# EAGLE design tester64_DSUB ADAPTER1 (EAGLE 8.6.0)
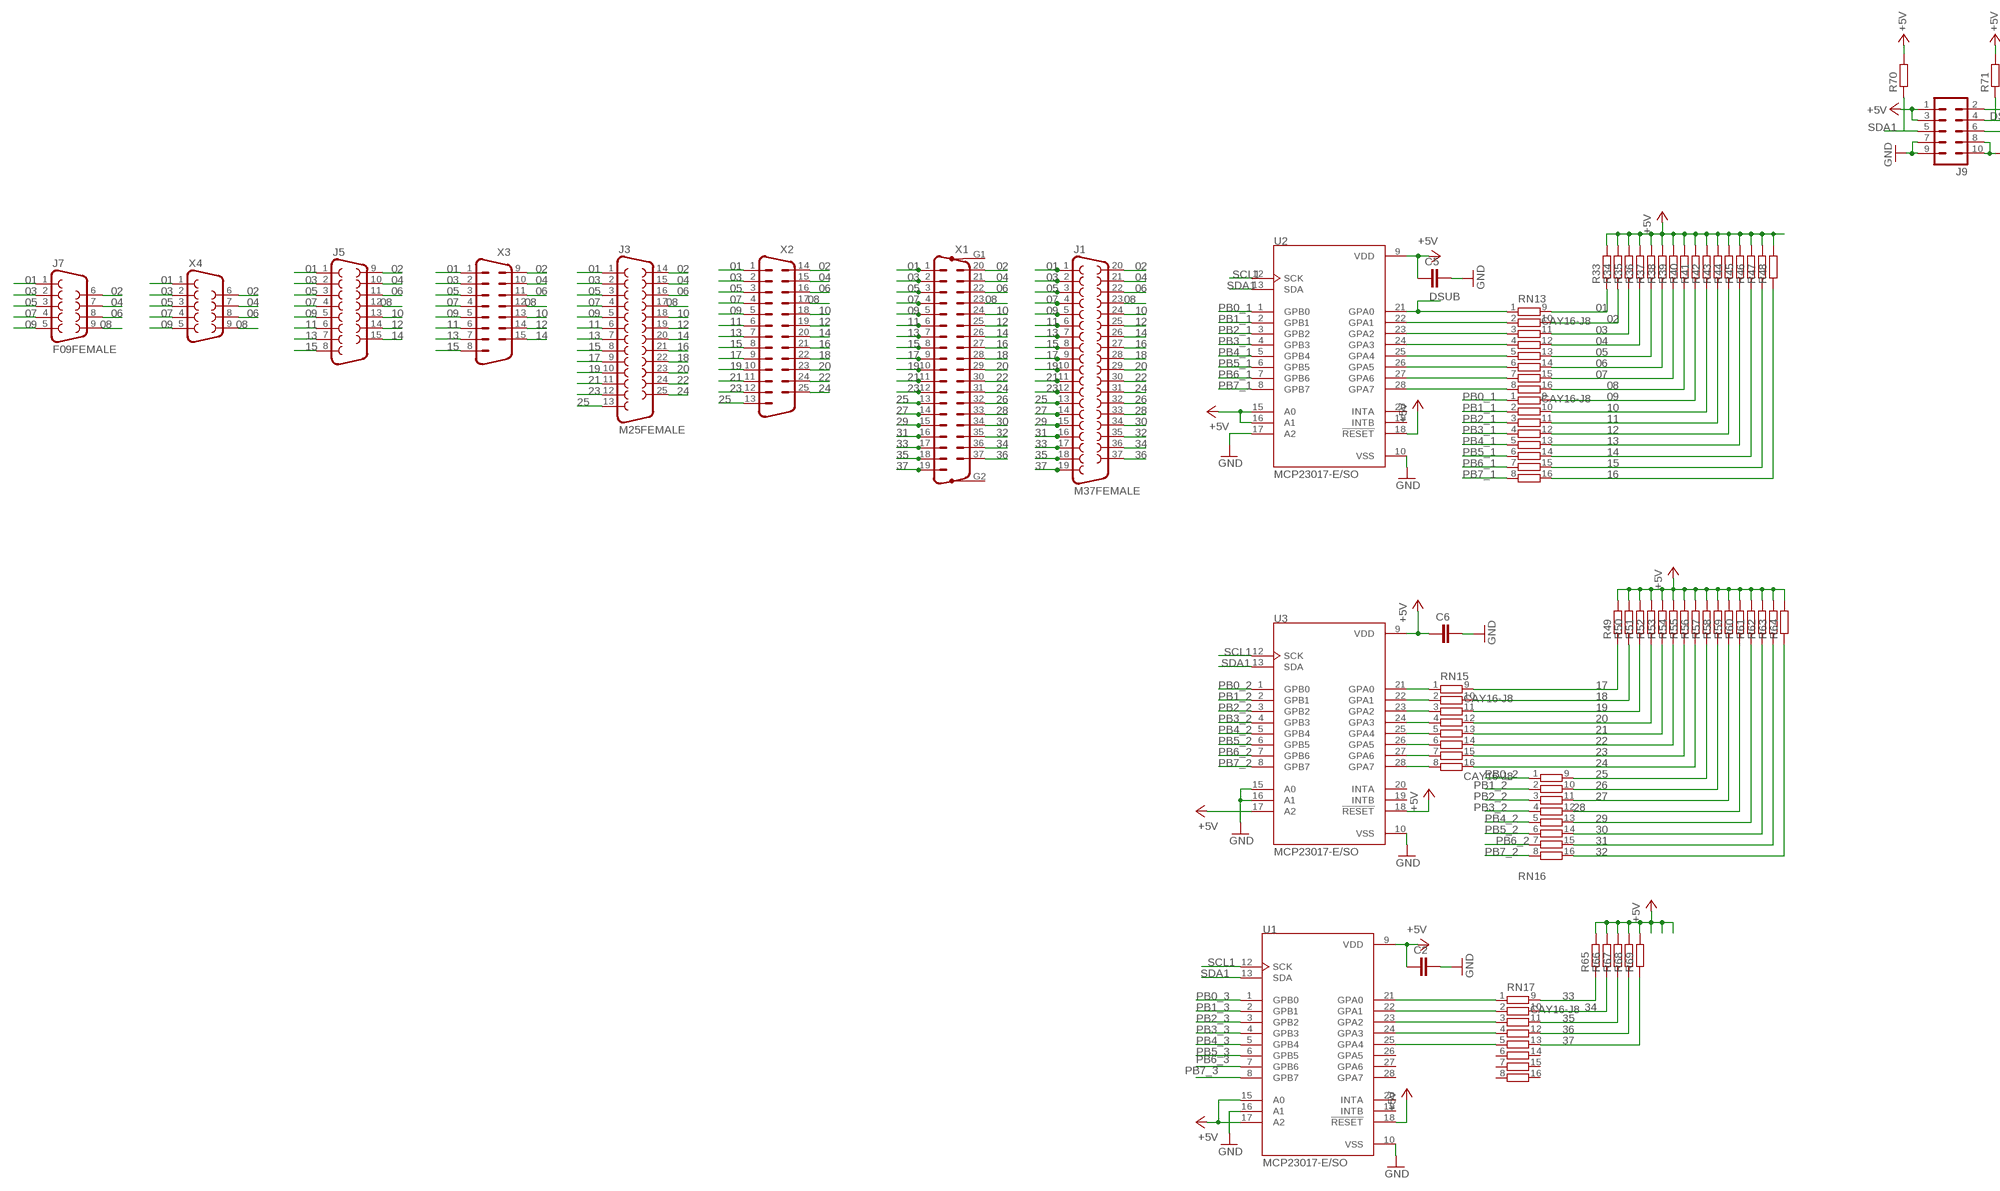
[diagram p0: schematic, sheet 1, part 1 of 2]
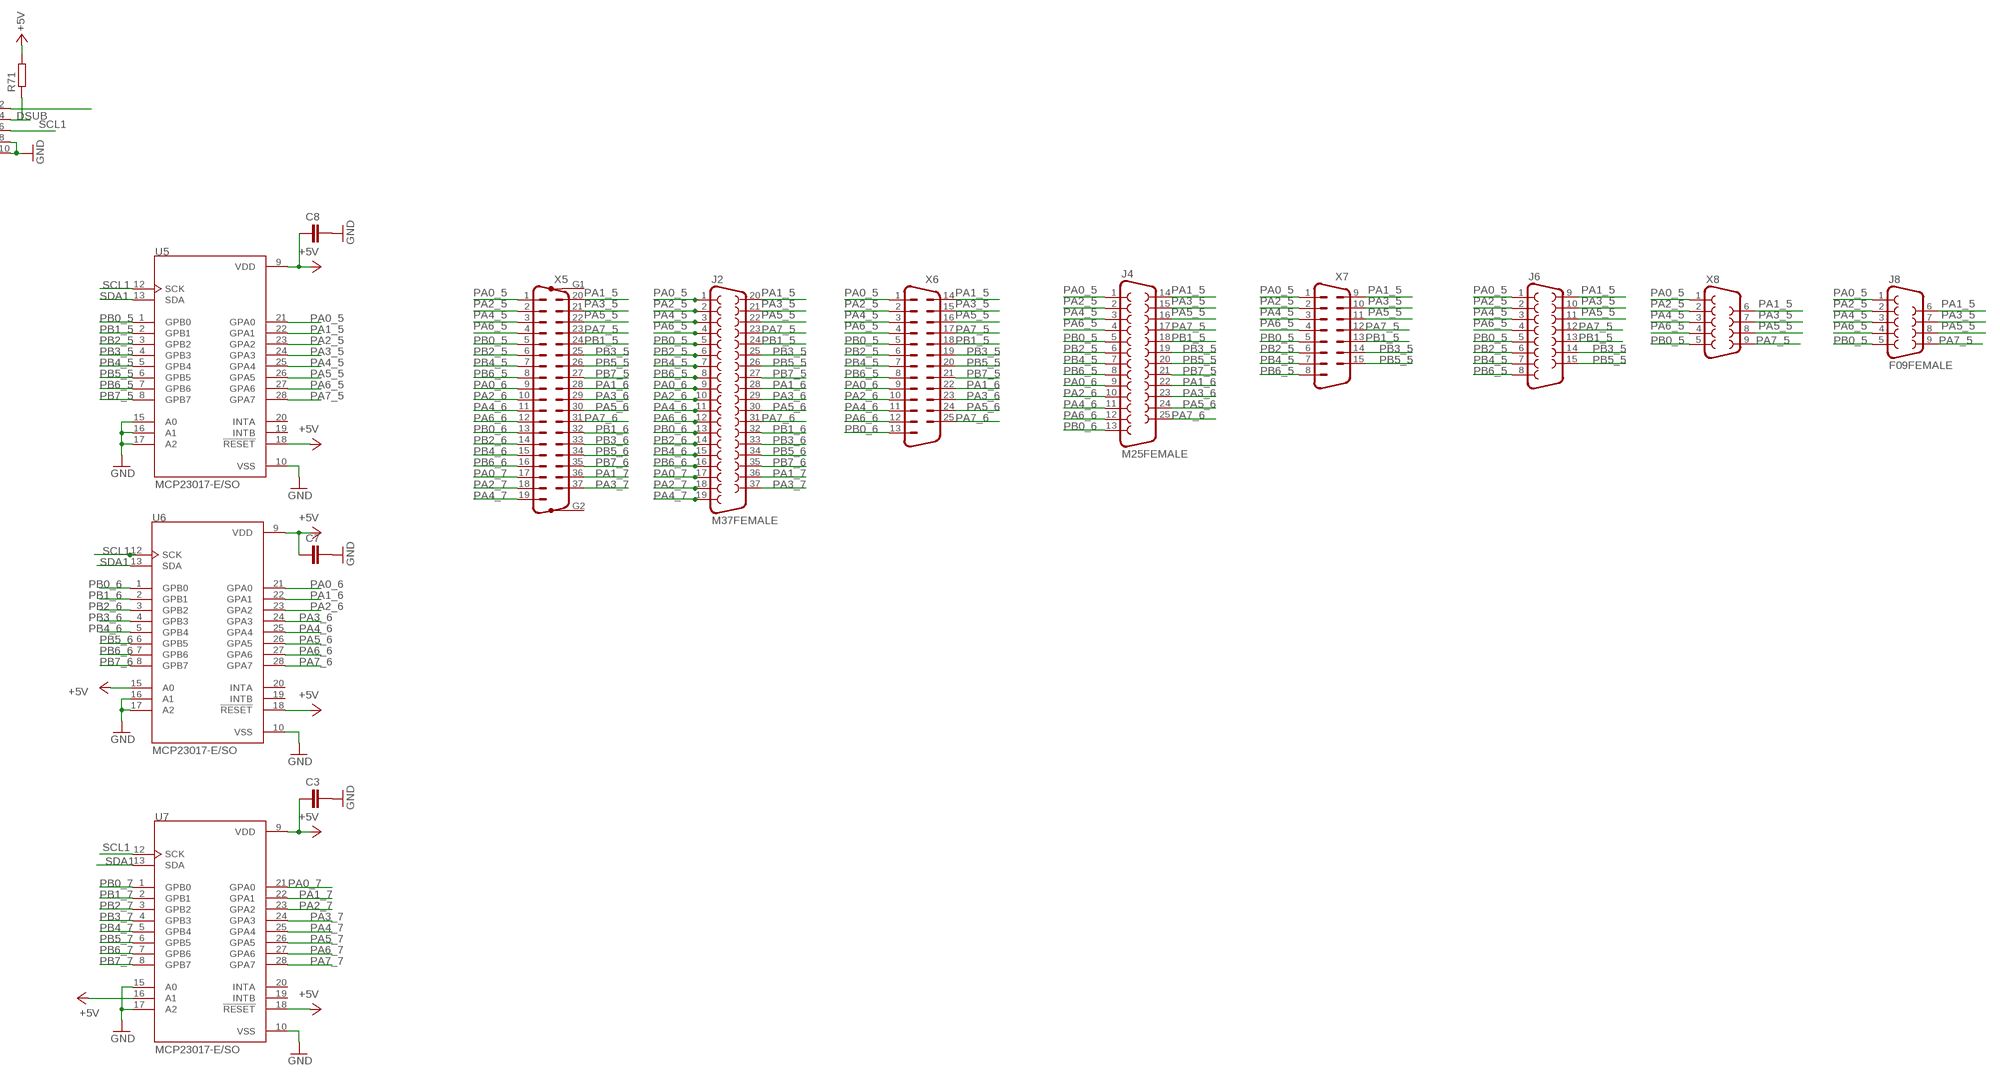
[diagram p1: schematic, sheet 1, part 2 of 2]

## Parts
C2  C-EUC0603  [C0603]
C3  C-EUC0603  [C0603]
C5  C-EUC0603  [C0603]
C6  C-EUC0603  [C0603]
C7  C-EUC0603  [C0603]
C8  C-EUC0603  [C0603]
J1  M37FEMALE  [M37FEMALE]
J2  M37FEMALE  [M37FEMALE]
J3  M25FEMALE  [M25FEMALE]
J4  M25FEMALE  [M25FEMALE]
J5  F15FEMALE  [M15FEMALE]
J6  F15FEMALE  [M15FEMALE]
J7  F09FEMALE  [FO9FEMALE]
J8  F09FEMALE  [FO9FEMALE]
J9  ML10  [ML10]
R33  R-EU_R0402  [R0402]
R34  R-EU_R0402  [R0402]
R35  R-EU_R0402  [R0402]
R36  R-EU_R0402  [R0402]
R37  R-EU_R0402  [R0402]
R38  R-EU_R0402  [R0402]
R39  R-EU_R0402  [R0402]
R40  R-EU_R0402  [R0402]
R41  R-EU_R0402  [R0402]
R42  R-EU_R0402  [R0402]
R43  R-EU_R0402  [R0402]
R44  R-EU_R0402  [R0402]
R45  R-EU_R0402  [R0402]
R46  R-EU_R0402  [R0402]
R47  R-EU_R0402  [R0402]
R48  R-EU_R0402  [R0402]
R49  R-EU_R0402  [R0402]
R50  R-EU_R0402  [R0402]
R51  R-EU_R0402  [R0402]
R52  R-EU_R0402  [R0402]
R53  R-EU_R0402  [R0402]
R54  R-EU_R0402  [R0402]
R55  R-EU_R0402  [R0402]
R56  R-EU_R0402  [R0402]
R57  R-EU_R0402  [R0402]
R58  R-EU_R0402  [R0402]
R59  R-EU_R0402  [R0402]
R60  R-EU_R0402  [R0402]
R61  R-EU_R0402  [R0402]
R62  R-EU_R0402  [R0402]
R63  R-EU_R0402  [R0402]
R64  R-EU_R0402  [R0402]
R65  R-EU_R0402  [R0402]
R66  R-EU_R0402  [R0402]
R67  R-EU_R0402  [R0402]
R68  R-EU_R0402  [R0402]
R69  R-EU_R0402  [R0402]
R70  R-EU_R0805  [R0805]
R71  R-EU_R0805  [R0805]
RN13  CAY16-J8  [CAY16Y8]
RN14  CAY16-J8  [CAY16Y8]
RN15  CAY16-J8  [CAY16Y8]
RN16  CAY16-J8  [CAY16Y8]
RN17  CAY16-J8  [CAY16Y8]
U1  MCP23017-E/SO  [SOIC127P1030X265-28N]
U2  MCP23017-E/SO  [SOIC127P1030X265-28N]
U3  MCP23017-E/SO  [SOIC127P1030X265-28N]
U5  MCP23017-E/SO  [SOIC127P1030X265-28N]
U6  MCP23017-E/SO  [SOIC127P1030X265-28N]
U7  MCP23017-E/SO  [SOIC127P1030X265-28N]
X1  M37VP  [M37VP]
X2  M25VP  [M25VP]
X3  M15V  [M15V]
X4  F09VP  [F09VP]
X5  M37VP  [M37VP]
X6  M25VP  [M25VP]
X7  M15V  [M15V]
X8  F09VP  [F09VP]

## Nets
01: J1.1 J3.1 J5.1 J7.1 R33.1 RN13.9 X1.1 X2.1 X3.1 X4.1
02: J1.20 J3.14 J5.9 J7.6 R34.1 RN13.10 X1.20 X2.14 X3.9 X4.6
03: J1.2 J3.2 J5.2 J7.2 R35.1 RN13.11 X1.2 X2.2 X3.2 X4.2
04: J1.21 J3.15 J5.10 J7.7 R36.1 RN13.12 X1.21 X2.15 X3.10 X4.7
05: J1.3 J3.3 J5.3 J7.3 R37.1 RN13.13 X1.3 X2.3 X3.3 X4.3
06: J1.22 J3.16 J5.11 J7.8 R38.1 RN13.14 X1.22 X2.16 X3.11 X4.8
07: J1.4 J3.4 J5.4 J7.4 R39.1 RN13.15 X1.4 X2.4 X3.4 X4.4
08: J1.23 J3.17 J5.12 J7.9 R40.1 RN13.16 X1.23 X2.17 X3.12 X4.9
09: J1.5 J3.5 J5.5 J7.5 R41.1 RN14.9 X1.5 X2.5 X3.5 X4.5
10: J1.24 J3.18 J5.13 R42.1 RN14.10 X1.24 X2.18 X3.13
11: J1.6 J3.6 J5.6 R43.1 RN14.11 X1.6 X2.6 X3.6
12: J1.25 J3.19 J5.14 R44.1 RN14.12 X1.25 X2.19 X3.14
13: J1.7 J3.7 J5.7 R45.1 RN14.13 X1.7 X2.7 X3.7
14: J1.26 J3.20 J5.15 R46.1 RN14.14 X1.26 X2.20 X3.15
15: J1.8 J3.8 J5.8 R47.1 RN14.15 X1.8 X2.8 X3.8
16: J1.27 J3.21 R48.1 RN14.16 X1.27 X2.21
17: J1.9 J3.9 R49.1 RN15.9 X1.9 X2.9
18: J1.28 J3.22 R50.1 RN15.10 X1.28 X2.22
19: J1.10 J3.10 R51.1 RN15.11 X1.10 X2.10
20: J1.29 J3.23 R52.1 RN15.12 X1.29 X2.23
21: J1.11 J3.11 R53.1 RN15.13 X1.11 X2.11
22: J1.30 J3.24 R54.1 RN15.14 X1.30 X2.24
23: J1.12 J3.12 R55.1 RN15.15 X1.12 X2.12
24: J1.31 J3.25 R56.1 RN15.16 X1.31 X2.25
25: J1.13 J3.13 R57.1 RN16.9 X1.13 X2.13
26: J1.32 R58.1 RN16.10 X1.32
27: J1.14 R59.1 RN16.11 X1.14
28: J1.33 R60.1 RN16.12 X1.33
29: J1.15 R61.1 RN16.13 X1.15
30: J1.34 R62.1 RN16.14 X1.34
31: J1.16 R63.1 RN16.15 X1.16
32: J1.35 R64.1 RN16.16 X1.35
33: J1.17 R65.1 RN17.9 X1.17
34: J1.36 R66.1 RN17.10 X1.36
35: J1.18 R67.1 RN17.11 X1.18
36: J1.37 R68.1 RN17.12 X1.37
37: J1.19 R69.1 RN17.13 X1.19
+5V: C2.2 C3.2 C5.2 C6.2 C7.2 C8.2 J9.1 J9.3 R33.2 R34.2 R35.2 R36.2 R37.2 R38.2 R39.2 R40.2 R41.2 R42.2 R43.2 R44.2 R45.2 R46.2 R47.2 R48.2 R49.2 R50.2 R51.2 R52.2 R53.2 R54.2 R55.2 R56.2 R57.2 R58.2 R59.2 R60.2 R61.2 R62.2 R63.2 R64.2 R65.2 R66.2 R67.2 R68.2 R69.2 R70.2 R71.2 U1.9(VDD) U1.15(A0) U1.17(A2) U1.18(!RESET) U2.9(VDD) U2.15(A0) U2.16(A1) U2.18(!RESET) U3.9(VDD) U3.17(A2) U3.18(!RESET) U5.9(VDD) U5.18(!RESET) U6.9(VDD) U6.15(A0) U6.18(!RESET) U7.9(VDD) U7.16(A1) U7.18(!RESET)
DSUB: J9.4 R71.1 RN13.1 U2.21(GPA0)
GND: C2.1 C3.1 C5.1 C6.1 C7.1 C8.1 J9.7 J9.8 J9.9 J9.10 U1.10(VSS) U1.16(A1) U2.10(VSS) U2.17(A2) U3.10(VSS) U3.15(A0) U3.16(A1) U5.10(VSS) U5.15(A0) U5.16(A1) U5.17(A2) U6.10(VSS) U6.16(A1) U6.17(A2) U7.10(VSS) U7.15(A0) U7.17(A2)
N$2: RN13.2 U2.22(GPA1)
N$3: RN13.3 U2.23(GPA2)
N$4: RN13.4 U2.24(GPA3)
N$5: RN13.5 U2.25(GPA4)
N$6: RN13.6 U2.26(GPA5)
N$7: RN13.7 U2.27(GPA6)
N$8: RN13.8 U2.28(GPA7)
N$9: RN15.1 U3.21(GPA0)
N$10: RN15.2 U3.22(GPA1)
N$11: RN15.3 U3.23(GPA2)
N$12: RN15.4 U3.24(GPA3)
N$13: RN15.5 U3.25(GPA4)
N$14: RN15.6 U3.26(GPA5)
N$15: RN15.7 U3.27(GPA6)
N$16: RN15.8 U3.28(GPA7)
N$28: RN17.1 U1.21(GPA0)
N$30: RN17.2 U1.22(GPA1)
N$31: RN17.3 U1.23(GPA2)
N$32: RN17.4 U1.24(GPA3)
N$33: RN17.5 U1.25(GPA4)
N$73: J9.2
PA0_5: J2.1 J4.1 J6.1 J8.1 U5.21(GPA0) X5.1 X6.1 X7.1 X8.1
PA0_6: J2.9 J4.9 U6.21(GPA0) X5.9 X6.9
PA0_7: J2.17 U7.21(GPA0) X5.17
PA1_5: J2.20 J4.14 J6.9 J8.6 U5.22(GPA1) X5.20 X6.14 X7.9 X8.6
PA1_6: J2.28 J4.22 U6.22(GPA1) X5.28 X6.22
PA1_7: J2.36 U7.22(GPA1) X5.36
PA2_5: J2.2 J4.2 J6.2 J8.2 U5.23(GPA2) X5.2 X6.2 X7.2 X8.2
PA2_6: J2.10 J4.10 U6.23(GPA2) X5.10 X6.10
PA2_7: J2.18 U7.23(GPA2) X5.18
PA3_5: J2.21 J4.15 J6.10 J8.7 U5.24(GPA3) X5.21 X6.15 X7.10 X8.7
PA3_6: J2.29 J4.23 U6.24(GPA3) X5.29 X6.23
PA3_7: J2.37 U7.24(GPA3) X5.37
PA4_5: J2.3 J4.3 J6.3 J8.3 U5.25(GPA4) X5.3 X6.3 X7.3 X8.3
PA4_6: J2.11 J4.11 U6.25(GPA4) X5.11 X6.11
PA4_7: J2.19 U7.25(GPA4) X5.19
PA5_5: J2.22 J4.16 J6.11 J8.8 U5.26(GPA5) X5.22 X6.16 X7.11 X8.8
PA5_6: J2.30 J4.24 U6.26(GPA5) X5.30 X6.24
PA5_7: U7.26(GPA5)
PA6_5: J2.4 J4.4 J6.4 J8.4 U5.27(GPA6) X5.4 X6.4 X7.4 X8.4
PA6_6: J2.12 J4.12 U6.27(GPA6) X5.12 X6.12
PA6_7: U7.27(GPA6)
PA7_5: J2.23 J4.17 J6.12 J8.9 U5.28(GPA7) X5.23 X6.17 X7.12 X8.9
PA7_6: J2.31 J4.25 U6.28(GPA7) X5.31 X6.25
PA7_7: U7.28(GPA7)
PB0_1: RN14.1 U2.1(GPB0)
PB0_2: RN16.1 U3.1(GPB0)
PB0_3: U1.1(GPB0)
PB0_5: J2.5 J4.5 J6.5 J8.5 U5.1(GPB0) X5.5 X6.5 X7.5 X8.5
PB0_6: J2.13 J4.13 U6.1(GPB0) X5.13 X6.13
PB0_7: U7.1(GPB0)
PB1_1: RN14.2 U2.2(GPB1)
PB1_2: RN16.2 U3.2(GPB1)
PB1_3: U1.2(GPB1)
PB1_5: J2.24 J4.18 J6.13 U5.2(GPB1) X5.24 X6.18 X7.13
PB1_6: J2.32 U6.2(GPB1) X5.32
PB1_7: U7.2(GPB1)
PB2_1: RN14.3 U2.3(GPB2)
PB2_2: RN16.3 U3.3(GPB2)
PB2_3: U1.3(GPB2)
PB2_5: J2.6 J4.6 J6.6 U5.3(GPB2) X5.6 X6.6 X7.6
PB2_6: J2.14 U6.3(GPB2) X5.14
PB2_7: U7.3(GPB2)
PB3_1: RN14.4 U2.4(GPB3)
PB3_2: RN16.4 U3.4(GPB3)
PB3_3: U1.4(GPB3)
PB3_5: J2.25 J4.19 J6.14 U5.4(GPB3) X5.25 X6.19 X7.14
PB3_6: J2.33 U6.4(GPB3) X5.33
PB3_7: U7.4(GPB3)
PB4_1: RN14.5 U2.5(GPB4)
PB4_2: RN16.5 U3.5(GPB4)
PB4_3: U1.5(GPB4)
PB4_5: J2.7 J4.7 J6.7 U5.5(GPB4) X5.7 X6.7 X7.7
PB4_6: J2.15 U6.5(GPB4) X5.15
PB4_7: U7.5(GPB4)
PB5_1: RN14.6 U2.6(GPB5)
PB5_2: RN16.6 U3.6(GPB5)
PB5_3: U1.6(GPB5)
PB5_5: J2.26 J4.20 J6.15 U5.6(GPB5) X5.26 X6.20 X7.15
PB5_6: J2.34 U6.6(GPB5) X5.34
PB5_7: U7.6(GPB5)
PB6_1: RN14.7 U2.7(GPB6)
PB6_2: RN16.7 U3.7(GPB6)
PB6_3: U1.7(GPB6)
PB6_5: J2.8 J4.8 J6.8 U5.7(GPB6) X5.8 X6.8 X7.8
PB6_6: J2.16 U6.7(GPB6) X5.16
PB6_7: U7.7(GPB6)
PB7_1: RN14.8 U2.8(GPB7)
PB7_2: RN16.8 U3.8(GPB7)
PB7_3: U1.8(GPB7)
PB7_5: J2.27 J4.21 U5.8(GPB7) X5.27 X6.21
PB7_6: J2.35 U6.8(GPB7) X5.35
PB7_7: U7.8(GPB7)
SCL1: J9.6 U1.12(SCK) U2.12(SCK) U3.12(SCK) U5.12(SCK) U6.12(SCK) U7.12(SCK)
SDA1: J9.5 R70.1 U1.13(SDA) U2.13(SDA) U3.13(SDA) U5.13(SDA) U6.13(SDA) U7.13(SDA)
Unconnected: RN17.6 RN17.7 RN17.8 RN17.14 RN17.15 RN17.16 U1.19(INTB) U1.20(INTA) U1.26(GPA5) U1.27(GPA6) U1.28(GPA7) U2.19(INTB) U2.20(INTA) U3.19(INTB) U3.20(INTA) U5.19(INTB) U5.20(INTA) U6.19(INTB) U6.20(INTA) U7.19(INTB) U7.20(INTA) X1.G1 X1.G2 X2.G1 X2.G2 X5.G1 X5.G2 X6.G1 X6.G2

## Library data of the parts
C2 C3 C5-C8 = rcl:C-EU: CAPACITOR, European symbol
J1 J2 = con-subd:M37FEMALE
J3 J4 = con-subd:M25FEMALE
J5 J6 = con-subd:F15FEMALE
J7 J8 = con-subd:F09FEMALE
J9 = con-harting-ml:ML10: HARTING; OC_FARNELL: unknown; OC_NEWARK: unknown
R33-R71 = rcl:R-EU_: RESISTOR, European symbol
RN13-RN17 = resistor-dil:CAY16-J8
U1-U3 U5-U7 = MCP23017-E_SO:MCP23017-E/SO: MCP23017 Series 5.5 V 1.7 MHz SMT 16-Bit I2C I/O Expander - SOIC-28 Check availability; AVAILABILITY: In Stock; CHECK_PRICES: https://www.snapeda.com/parts/MCP23017-E/SO/Microchip/view-part/?ref=eda; DESCRIPTION: I/O Port Expander, 16-Bit, I2C I'face, SOIC-28 | Microchip Technology Inc. MCP23017-E/SO; MF: Microchip; MP: MCP23017-E/SO; PACKAGE: SOIC-28 Microchip; PRICE: None; PURCHASE-URL: https://www.snapeda.com/api/url_track_click_mouser/?unipart_id=48467&manufacturer=Microchip&part_name=MCP23017-E/SO&search_term=mcp23017; SNAPEDA_LINK: https://www.snapeda.com/parts/MCP23017-E/SO/Microchip/view-part/?ref=snap
X1 X5 = con-subd:M37VP: SUB-D; OC_FARNELL: unknown; OC_NEWARK: unknown
X2 X6 = con-subd:M25VP: SUB-D; OC_FARNELL: unknown; OC_NEWARK: unknown
X3 X7 = con-subd:M15: SUB-D; OC_FARNELL: unknown; OC_NEWARK: unknown
X4 X8 = con-subd:F09: SUB-D; OC_FARNELL: unknown; OC_NEWARK: unknown

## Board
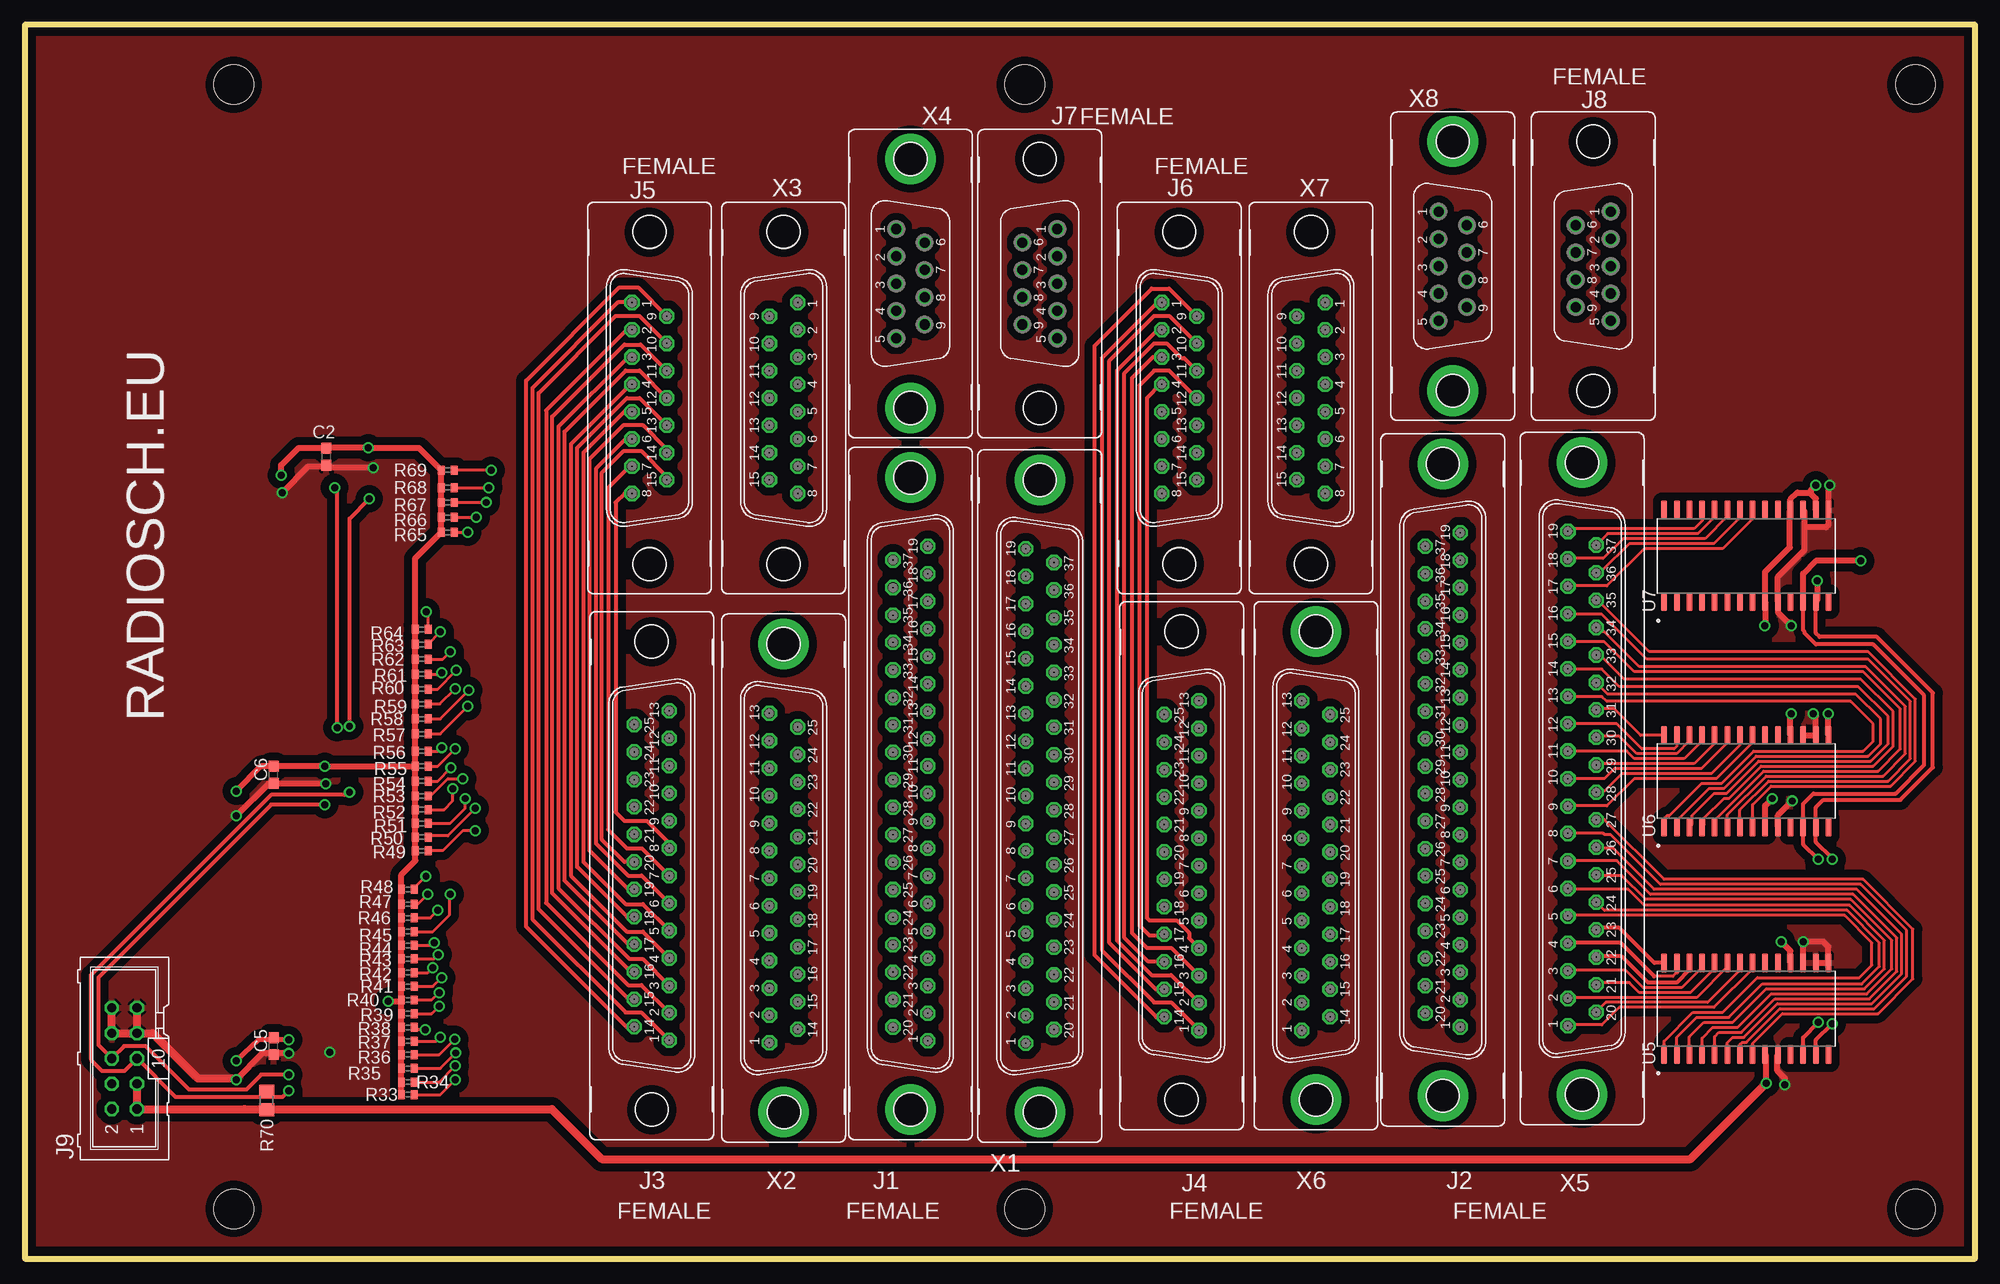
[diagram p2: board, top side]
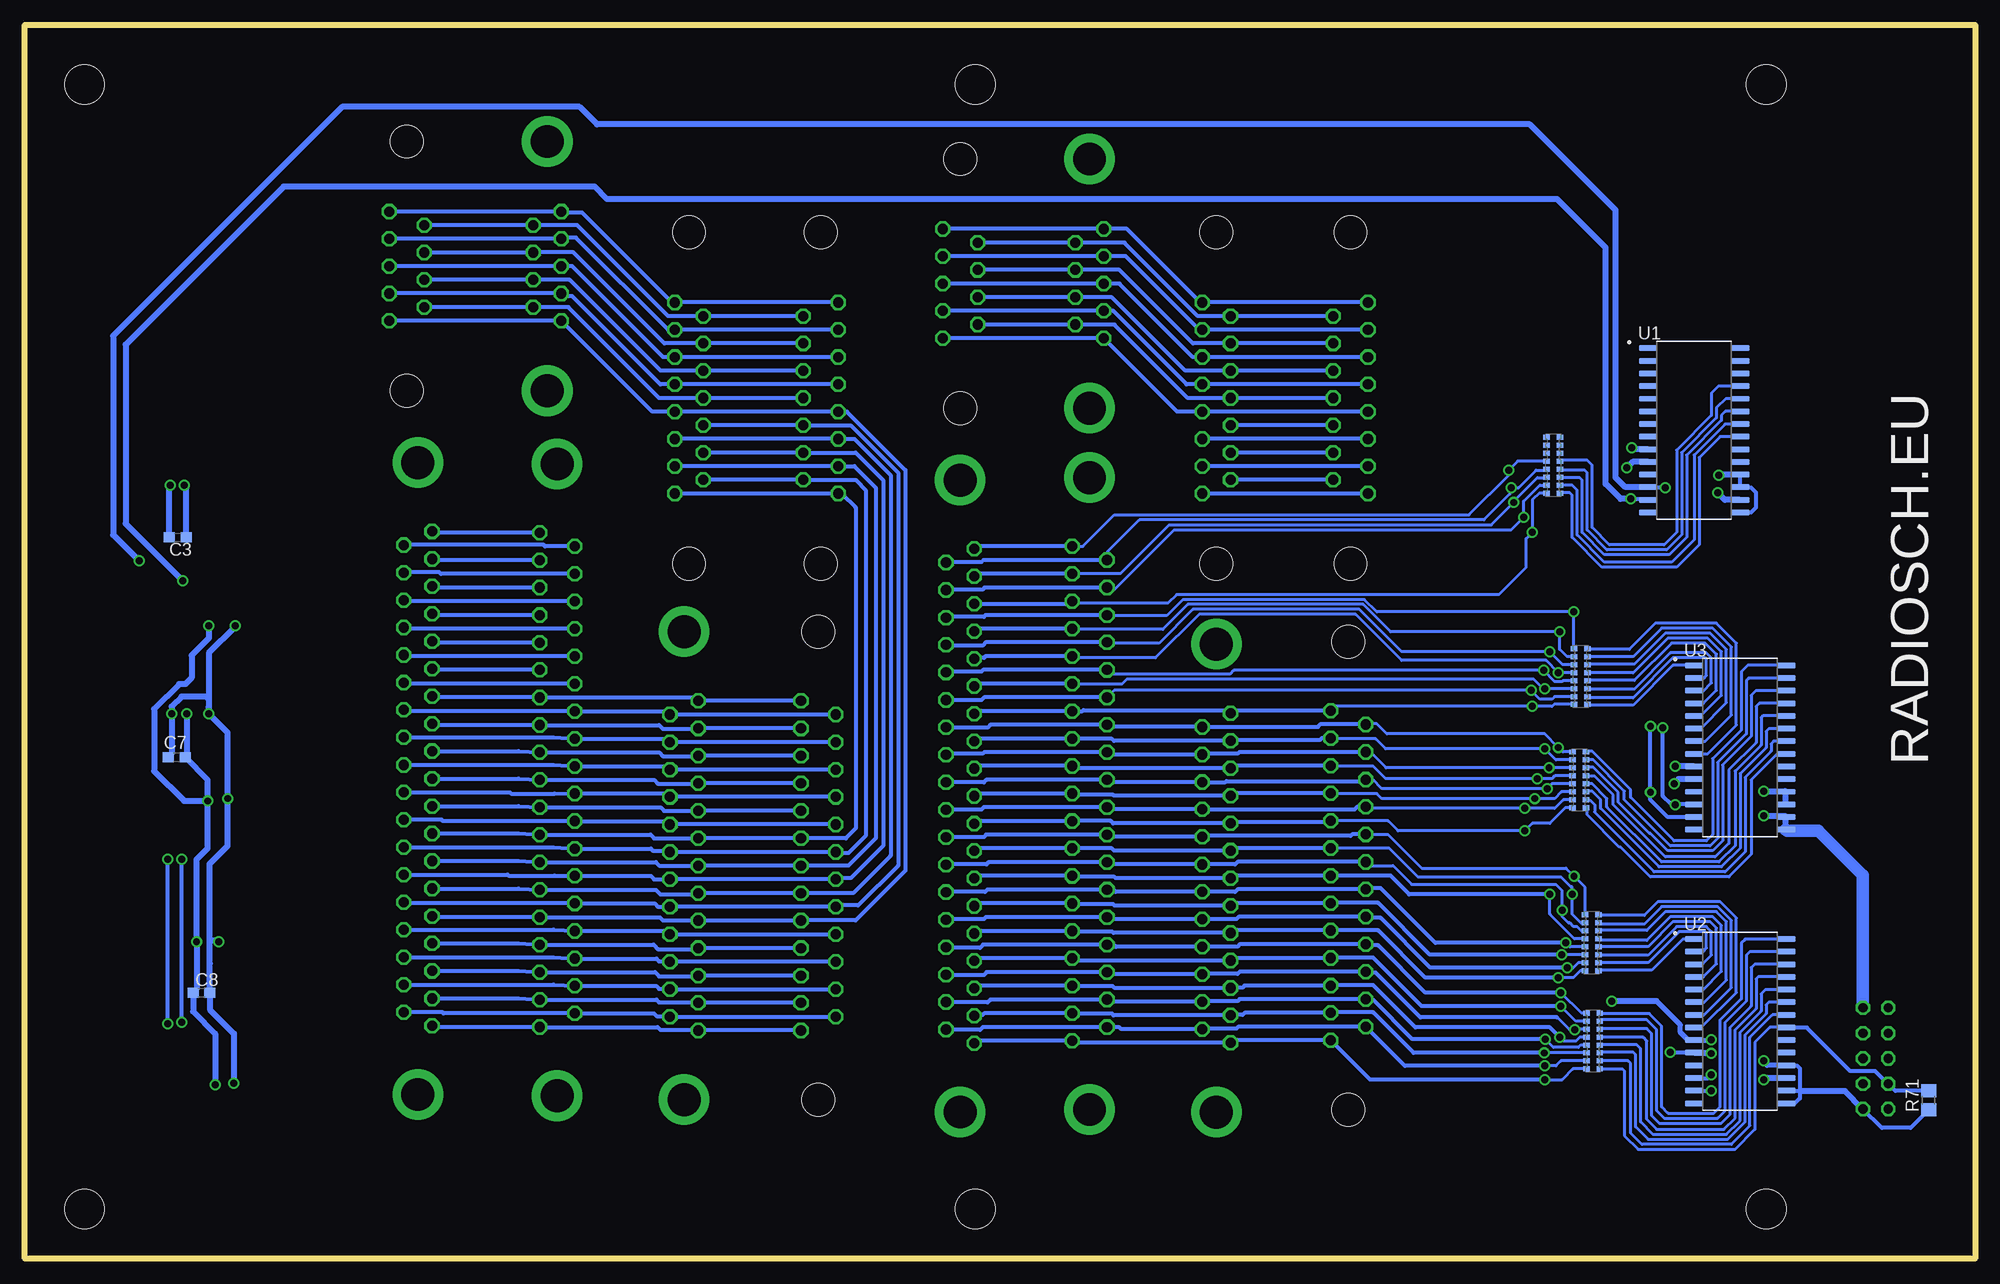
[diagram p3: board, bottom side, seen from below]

Size 196 x 124 mm. Coordinates in mm from the lower left corner, seen from the top.
Outline: 0,0 196,0 196,124 0,124 0,0
Copper layers (1*16): Top 0.035mm / dielectric 1.5mm / Bottom 0.035mm
Design rules "default *": minimum track width 10mil, minimum drill 24mil, track to track 5mil, track to pad 5mil, pad to pad 5mil, via to via 5mil, smd to smd 5mil, copper to edge 20mil, drill to drill 8mil, minimum pad ring 10mil, minimum via ring 8mil, stop-mask expansion 4mil, vias tented up to drill 0mil, thermal gap 10mil
Holes 4 mm at 21,5 190,5 21,118 190,118 100.5,118 100.5,5

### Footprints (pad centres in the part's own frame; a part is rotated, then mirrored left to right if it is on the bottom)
C0603 = smd 1.1 x 1: 1 -0.85,0; 2 0.85,0
M37FEMALE = drill 1.016 octagon: 1 56.591,1.753; 2 53.848,1.753; 3 51.079,1.753; 4 48.311,1.753; 5 45.568,1.753; 6 42.799,1.753; 7 40.03,1.753; 8 37.262,1.753; 9 34.519,1.753; 10 31.75,1.753; 11 28.981,1.753; 12 26.238,1.753; 13 23.47,1.753; 14 20.701,1.753; 15 17.958,1.753; 16 15.189,1.753; 17 12.421,1.753; 18 9.677,1.753; 19 6.909,1.753; 20 55.22,-1.753; 21 52.451,-1.753; 22 49.708,-1.753; 23 46.939,-1.753; 24 44.171,-1.753; 25 41.402,-1.753; 26 38.659,-1.753; 27 35.89,-1.753; 28 33.122,-1.753; 29 30.378,-1.753; 30 27.61,-1.753; 31 24.841,-1.753; 32 22.098,-1.753; 33 19.329,-1.753; 34 16.561,-1.753; 35 13.818,-1.753; 36 11.049,-1.753; 37 8.28,-1.753 | drill 3.302 pad 5.08: G1 0,0; G2 63.5,0
M25FEMALE = drill 1.016 octagon: 1 16.561,1.753; 2 13.792,1.753; 3 11.049,1.753; 4 8.28,1.753; 5 5.512,1.753; 6 2.769,1.753; 7 0,1.753; 8 -2.769,1.753; 9 -5.512,1.753; 10 -8.28,1.753; 11 -11.049,1.753; 12 -13.792,1.753; 13 -16.561,1.753; 14 15.189,-1.753; 15 12.421,-1.753; 16 9.652,-1.753; 17 6.909,-1.753; 18 4.14,-1.753; 19 1.372,-1.753; 20 -1.372,-1.753; 21 -4.14,-1.753; 22 -6.909,-1.753; 23 -9.652,-1.753; 24 -12.421,-1.753; 25 -15.189,-1.753 | hole 3.302: 23.52,0; -23.52,0
M15FEMALE = drill 1.016 octagon: 1 9.601,0.483; 2 6.858,0.483; 3 4.115,0.483; 4 1.372,0.483; 5 -1.372,0.483; 6 -4.115,0.483; 7 -6.858,0.483; 8 -9.601,0.483; 9 8.23,-3.023; 10 5.486,-3.023; 11 2.743,-3.023; 12 0,-3.023; 13 -2.743,-3.023; 14 -5.486,-3.023; 15 -8.23,-3.023 | hole 3.302: 16.662,-1.27; -16.662,-1.27
FO9FEMALE = drill 1.016 octagon: 1 -5.486,1.753; 2 -2.743,1.753; 3 0,1.753; 4 2.743,1.753; 5 5.486,1.753; 6 -4.115,-1.753; 7 -1.372,-1.753; 8 1.372,-1.753; 9 4.115,-1.753 | hole 3.302: -12.522,0; 12.522,0
ML10 = drill 0.914 octagon: 1 -5.08,-1.27; 2 -5.08,1.27; 3 -2.54,-1.27; 4 -2.54,1.27; 5 0,-1.27; 6 0,1.27; 7 2.54,-1.27; 8 2.54,1.27; 9 5.08,-1.27; 10 5.08,1.27
R0402 = smd 0.7 x 0.9: 1 -0.65,0; 2 0.65,0
R0805 = smd 1.3 x 1.5: 1 -0.95,0; 2 0.95,0
CAY16Y8 = smd 0.5 x 0.65: 1 -3.8,0.225; 2 -3,0.225; 3 -2.2,0.225; 4 -1.4,0.225; 5 -0.6,0.225; 6 0.2,0.225; 7 1,0.225; 8 1.8,0.225; 9 -3.8,1.575; 10 -3,1.575; 11 -2.2,1.575; 12 -1.4,1.575; 13 -0.6,1.575; 14 0.2,1.575; 15 1,1.575; 16 1.8,1.575
SOIC127P1030X265-28N = smd 1.9 x 0.6: 1 -4.605,8.255; 2 -4.605,6.985; 3 -4.605,5.715; 4 -4.605,4.445; 5 -4.605,3.175; 6 -4.605,1.905; 7 -4.605,0.635; 8 -4.605,-0.635; 9 -4.605,-1.905; 10 -4.605,-3.175; 11 -4.605,-4.445; 12 -4.605,-5.715; 13 -4.605,-6.985; 14 -4.605,-8.255; 15 4.605,-8.255; 16 4.605,-6.985; 17 4.605,-5.715; 18 4.605,-4.445; 19 4.605,-3.175; 20 4.605,-1.905; 21 4.605,-0.635; 22 4.605,0.635; 23 4.605,1.905; 24 4.605,3.175; 25 4.605,4.445; 26 4.605,5.715; 27 4.605,6.985; 28 4.605,8.255
M37VP = drill 1.016 octagon: 1 -24.841,1.422; 2 -22.098,1.422; 3 -19.329,1.422; 4 -16.561,1.422; 5 -13.818,1.422; 6 -11.049,1.422; 7 -8.28,1.422; 8 -5.512,1.422; 9 -2.769,1.422; 10 0,1.422; 11 2.769,1.422; 12 5.512,1.422; 13 8.28,1.422; 14 11.049,1.422; 15 13.792,1.422; 16 16.561,1.422; 17 19.329,1.422; 18 22.073,1.422; 19 24.841,1.422; 20 -23.47,-1.422; 21 -20.701,-1.422; 22 -17.958,-1.422; 23 -15.189,-1.422; 24 -12.421,-1.422; 25 -9.652,-1.422; 26 -6.909,-1.422; 27 -4.14,-1.422; 28 -1.372,-1.422; 29 1.372,-1.422; 30 4.14,-1.422; 31 6.909,-1.422; 32 9.652,-1.422; 33 12.421,-1.422; 34 15.189,-1.422; 35 17.932,-1.422; 36 20.701,-1.422; 37 23.47,-1.422 | drill 3.302 pad 5.08: G1 -31.75,0; G2 31.75,0
M25VP = drill 1.016 octagon: 1 -16.561,1.422; 2 -13.792,1.422; 3 -11.049,1.422; 4 -8.28,1.422; 5 -5.512,1.422; 6 -2.769,1.422; 7 0,1.422; 8 2.769,1.422; 9 5.512,1.422; 10 8.28,1.422; 11 11.049,1.422; 12 13.792,1.422; 13 16.561,1.422; 14 -15.189,-1.422; 15 -12.421,-1.422; 16 -9.652,-1.422; 17 -6.909,-1.422; 18 -4.14,-1.422; 19 -1.372,-1.422; 20 1.372,-1.422; 21 4.14,-1.422; 22 6.909,-1.422; 23 9.652,-1.422; 24 12.421,-1.422; 25 15.189,-1.422 | drill 3.302 pad 5.08: G1 -23.52,0; G2 23.52,0
M15V = drill 1.016 octagon: 1 -9.601,1.422; 2 -6.858,1.422; 3 -4.115,1.422; 4 -1.372,1.422; 5 1.372,1.422; 6 4.115,1.422; 7 6.858,1.422; 8 9.601,1.422; 9 -8.23,-1.422; 10 -5.486,-1.422; 11 -2.743,-1.422; 12 0,-1.422; 13 2.743,-1.422; 14 5.486,-1.422; 15 8.23,-1.422 | hole 3.302: 16.662,0; -16.662,0
F09VP = drill 1.016 octagon: 1 5.486,1.422; 2 2.743,1.422; 3 0,1.422; 4 -2.743,1.422; 5 -5.486,1.422; 6 4.115,-1.422; 7 1.372,-1.422; 8 -1.372,-1.422; 9 -4.115,-1.422 | drill 3.302 pad 5.08: G1 -12.522,0; G2 12.522,0

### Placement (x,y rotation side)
C2  30.31,80.58 90 top
C3  180.62,72.5 0 bottom
C5  25,21.38 90 top
C6  25,48.62 90 top
C7  180.75,50.38 180 bottom
C8  178.25,26.75 0 bottom
J1  89,78.5 270 top
J2  142.5,79.88 270 top
J3  63,38.5 270 top
J4  116.25,39.5 270 top
J5  61.5,86.5 90 top
J6  114.75,86.5 90 top
J7  102,98 270 top
J8  157.62,99.75 270 top
J9  10,20.12 90 top
R33  38.5,16.5 180 top
R34  38.5,17.75 180 top
R35  38.5,19.12 180 top
R36  38.5,20.5 180 top
R37  38.5,21.88 180 top
R38  38.5,23.25 180 top
R39  38.5,24.62 180 top
R40  38.5,26 180 top
R41  38.5,27.38 180 top
R42  38.5,28.75 180 top
R43  38.5,30.12 180 top
R44  38.5,31.5 180 top
R45  38.5,32.88 180 top
R46  38.5,34.25 180 top
R47  38.5,35.62 180 top
R48  38.5,37.12 180 top
R49  39.88,41 180 top
R50  39.88,42.38 180 top
R51  39.88,43.75 180 top
R52  39.88,45.12 180 top
R53  39.88,46.5 180 top
R54  39.88,48 180 top
R55  39.88,49.5 180 top
R56  39.88,51 180 top
R57  39.88,52.75 180 top
R58  39.88,54.25 180 top
R59  39.88,55.75 180 top
R60  39.88,57.25 180 top
R61  39.88,58.75 180 top
R62  39.88,60.25 180 top
R63  39.88,61.75 180 top
R64  39.88,63.25 180 top
R65  42.5,73 180 top
R66  42.5,74.5 180 top
R67  42.5,76 180 top
R68  42.5,77.5 180 top
R69  42.5,79.25 180 top
R70  24.3,15.9 270 top
R71  4.67,15.93 270 bottom
RN13  37.5,22.88 90 bottom
RN14  37.62,32.75 90 bottom
RN15  38.88,49.12 90 bottom
RN16  38.75,59.5 90 bottom
RN17  41.5,80.75 90 bottom
U1  28.25,83.25 0 bottom
U2  23.62,23.88 0 bottom
U3  23.62,51.38 0 bottom
U5  173,25.12 90 top
U6  173,48 90 top
U7  173,70.62 90 top
X1  102,46.5 90 top
X2  76.25,38.25 90 top
X3  76.25,86.5 270 top
X4  89,98 90 top
X5  156.5,48.25 90 top
X6  129.75,39.5 90 top
X7  129.25,86.5 270 top
X8  143.5,99.75 90 top

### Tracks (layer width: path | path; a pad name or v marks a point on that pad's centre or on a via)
01  (via drill 0.7)
  Top 0.305: R33.1 41.75,16.5 v43.25,18
  Top 0.406: J5.1 59.6,96.1 51,87.5 51,34.12 60.38,24.75 61.94,24.75 J3.1
  Bottom 0.305: RN13.9 40.42,19.07 41.5,18 v43.25,18
  Bottom 0.406: v43.25,18 60.81,18 J3.1 74.58,21.94 X2.1 90.53,21.69 J1.1 100.33,21.91 X1.1 | J5.1 X3.1 77.85,96.1 85.25,103.5 87.56,103.5 X4.1 J7.1
02  (via drill 0.7)
  Top 0.305: R34.1 41.62,17.75 v43.25,19.38
  Top 0.406: J3.14 60.44,23.31 50.38,33.38 50.38,88.25 59.75,97.62 61.63,97.62 J5.9
  Bottom 0.305: RN13.10 41.62,19.88 42.12,19.38 v43.25,19.38 43.38,19.38
  Bottom 0.406: 43.38,19.38 57.31,19.38 J3.14 74.06,23.31 74.25,23.12 77.61,23.12 X2.14 85.81,23.06 86,23.25 87.22,23.25 J1.20 99.72,23.28 100,23 103.39,23 X1.20 | J5.9 X3.9 78.11,94.73 85.5,102.12 90.41,102.12 X4.6 J7.6
03  (via drill 0.7)
  Top 0.305: R35.1 41.75,19.12 v43.3,20.68
  Top 0.406: J5.2 60.48,93.36 52.38,85.25 52.38,35.75 60.62,27.5 61.96,27.5 J3.2
  Bottom 0.305: RN13.11 v43.3,20.68
  Bottom 0.406: v43.3,20.68 56.42,20.68 60.5,24.75 64.71,24.75 J3.2 73.42,24.71 73.62,24.5 74.78,24.5 X2.2 86.58,24.46 86.75,24.62 90.73,24.62 J1.2 99.6,24.65 99.75,24.5 100.48,24.5 X1.2 | J5.2 X3.2 77.98,93.36 85.38,100.75 X4.2 J7.2
04  (via drill 0.7)
  Top 0.305: R36.1 41.62,20.5 v43.19,22.06
  Top 0.406: J3.15 60.67,26.08 51.62,35.12 51.62,87 59.38,94.75 61.76,94.75 J5.10
  Bottom 0.305: v43.19,22.06 42.38,21.25 39.88,21.25 39.62,21.5 39.1,21.5 RN13.12
  Bottom 0.406: v43.19,22.06 56.56,22.06 60.5,26 61.17,26 J3.15 73.92,26.08 74.12,25.88 77.63,25.88 X2.15 87.03,25.83 J1.21 98.95,26.05 99.25,25.75 103.37,25.75 X1.21 | J5.10 X3.10 78.61,91.99 86,99.38 X4.7 J7.7
05  (via drill 0.7)
  Top 0.305: R37.1 41.35,21.88 v41.75,22.27
  Top 0.406: J5.3 60.62,90.61 53.62,83.62 53.62,37.25 60.75,30.12 62.08,30.12 J3.3
  Bottom 0.305: 41.9,22.27 v41.75,22.27 41.35,21.88 40.12,21.88 39.73,22.27 RN13.13
  Bottom 0.406: 41.9,22.27 41.9,22.4 42.75,23.25 56.25,23.25 60.5,27.5 64.7,27.5 J3.3 73.42,27.45 73.62,27.25 74.78,27.25 X2.3 86.45,27.2 86.62,27.38 90.71,27.38 J1.3 100.33,27.42 X1.3 | J5.3 X3.3 78.61,90.61 86,98 X4.3 J7.3
06  (via drill 0.7)
  Top 0.305: v40.25,23 39.4,23 R38.1
  Top 0.406: J3.16 60.9,28.85 53,36.75 53,84.62 60.25,91.88 61.89,91.88 J5.11
  Bottom 0.305: RN13.14 40.17,23.07 v40.25,23 40.75,23 42,24.25
  Bottom 0.406: 42,24.25 55.75,24.25 60.25,28.75 61.15,28.75 J3.16 73.9,28.85 74.12,28.62 77.64,28.62 X2.16 86.47,28.6 86.62,28.75 87.2,28.75 J1.22 99.33,28.79 99.62,28.5 103.38,28.5 X1.22 | J5.11 X3.11 79.37,89.24 86.75,96.62 X4.8 J7.8
07  (via drill 0.7)
  Top 0.305: R39.1 40.88,24.62 v41.62,25.38
  Top 0.406: J5.4 60.87,87.87 54.88,81.88 54.88,38.5 60.5,32.88 62.1,32.88 J3.4
  Bottom 0.305: RN13.15 40.12,23.88 v41.62,25.38
  Bottom 0.406: v41.62,25.38 55.62,25.38 60.5,30.25 64.72,30.25 J3.4 74.58,30.22 X2.4 90.53,29.97 J1.4 100.33,30.19 X1.4 | J5.4 77.12,87.87 77.12,87.88 X3.4 79.25,87.87 86.62,95.25 X4.4 J7.4
08  (via drill 0.7)
  Top 0.305: R40.1 40.88,26 v41.62,26.75
  Top 0.406: J3.17 60.66,31.59 54.25,38 54.25,83.12 60.38,89.25 61.77,89.25 J5.12
  Bottom 0.305: RN13.16 39.55,24.68 v41.62,26.75
  Bottom 0.406: v41.62,26.75 55.25,26.75 60,31.5 61.16,31.5 J3.17 73.91,31.59 74.12,31.38 77.64,31.38 X2.17 86.34,31.34 86.62,31.62 87.18,31.62 J1.23 99.69,31.56 100,31.25 103.36,31.25 X1.23 | J5.12 X3.12 79.12,86.5 86.5,93.88 90.41,93.88 X4.9 J7.9
09  (via drill 0.7)
  Top 0.305: R41.1 41,27.38 v41.88,28.25
  Top 0.406: J5.5 60.25,85.13 56.12,81 56.12,39.88 60.38,35.62 62.12,35.62 J3.5
  Bottom 0.305: RN14.9 39.67,28.95 40.38,28.25 v41.88,28.25
  Bottom 0.406: v41.88,28.25 55.25,28.25 60,33 J3.5 74.58,32.99 X2.5 86.61,32.74 86.75,32.88 90.69,32.88 J1.5 100.33,32.93 X1.5 | J5.5 X3.5 80.19,85.13 X4.5 J7.5
10  (via drill 0.7)
  Top 0.305: R42.1 40.5,28.75 v41,29.25
  Top 0.406: J3.18 60.52,34.36 55.5,39.38 55.5,81.5 60.5,86.5 61.78,86.5 J5.13
  Bottom 0.305: RN14.10 39.88,29.75 40.38,29.25 v41,29.25 41.62,29.25
  Bottom 0.406: 41.62,29.25 54.75,29.25 59.75,34.25 61.14,34.25 J3.18 74.02,34.36 74.25,34.12 77.66,34.12 X2.18 87.03,34.11 J1.24 99.42,34.33 99.62,34.12 103.38,34.12 X1.24 | J5.13 X3.13
11  (via drill 0.7)
  Top 0.305: R43.1 41.12,30.12 v41.55,30.55
  Top 0.406: J5.6 60.38,82.39 57.38,79.38 57.38,41.75 60.62,38.5 61.98,38.5 J3.6
  Bottom 0.305: RN14.11 v41.55,30.55
  Bottom 0.406: v41.55,30.55 54.8,30.55 60,35.75 64.73,35.75 J3.6 74.58,35.73 X2.6 86.48,35.48 86.62,35.62 90.68,35.62 J1.6 100.33,35.7 X1.6 | J5.6 X3.6
12  (via drill 0.7)
  Top 0.305: R44.1 40.88,31.5 v41.12,31.75
  Top 0.406: J5.14 64.52,81.35 62.12,83.75 60.12,83.75 56.75,80.38 56.75,41 60.62,37.13 J3.19
  Bottom 0.305: RN14.12 40.73,31.35 v41.12,31.75
  Bottom 0.406: v41.12,31.75 54.25,31.75 59.75,37.25 61.13,37.25 J3.19 74.12,37.13 74.38,36.88 X2.19 86.38,36.88 86.62,37.12 87.22,37.12 J1.25 99.28,37.1 99.5,36.88 103.39,36.88 X1.25 | J5.14 X3.14
13  (via drill 0.7)
  Top 0.305: R45.1 41,32.88 42.69,34.56 42.69,36.56 v42.75,36.62
  Top 0.406: J5.7 60.77,79.64 58.62,77.5 58.62,43.12 60.5,41.25 62,41.25 J3.7
  Bottom 0.305: RN14.13 40.27,32.15 42.75,34.62 v42.75,36.62
  Bottom 0.406: v42.75,36.62 56.88,36.62 58.75,38.5 J3.7 74.58,38.5 X2.7 86.38,38.25 86.5,38.38 90.66,38.38 J1.7 100.33,38.47 X1.7 | J5.7 X3.7
14  (via drill 0.7)
  Top 0.305: R46.1 40.75,34.25 v41.5,35
  Top 0.406: J5.15 64.52,78.6 62,81.12 60.12,81.12 58,79 58,42.12 60.25,39.87 J3.20
  Bottom 0.305: RN14.14 39.58,32.95 40,33.38 40.38,33.38 40.75,33.75 40.88,33.75 41.5,34.38 v41.5,35 41.5,37 42.12,37.62 56.62,37.62 58.5,39.5 60.88,39.5
  Bottom 0.406: 60.88,39.5 J3.20 74.13,39.87 74.38,39.62 X2.20 87.03,39.62 J1.26 99.16,39.84 99.38,39.62 103.39,39.62 X1.26 | J5.15 X3.15
15  (via drill 0.7)
  Top 0.305: R47.1 39.5,35.62 v40.5,36.62
  Top 0.406: J5.8 60.27,76.9 59.38,76 59.38,44.88 60.25,44 62.5,44 64.5,42 64.5,41.52 J3.8
  Bottom 0.305: RN14.15 39.62,33.75 40.5,34.62 v40.5,36.62 40.5,37.38 40.62,37.38 41.62,38.38 56,38.38 58.88,41.25 64.73,41.25 J3.8
  Bottom 0.406: J3.8 74.58,41.27 X2.8 86.52,41.02 86.75,41.25 J1.8 100.33,41.24 X1.8 | J5.8 X3.8
16  (via drill 0.7)
  Top 0.305: R48.1 39.15,37.27 v40.31,38.44
  Bottom 0.305: RN14.16 39.2,37.33 v40.31,38.44 41.12,39.25 55.62,39.25 59.02,42.64 J3.21
  Bottom 0.406: J3.21 62.61,42.64 62.75,42.5 77.56,42.5 X2.21 87.03,42.39 J1.27 99.39,42.61 99.62,42.38 103.41,42.38 X1.27
17  (via drill 0.7)
  Top 0.305: v45.25,43 44,43 42,41 R49.1
  Bottom 0.305: RN15.9 41.17,45.33 42.75,43.75 44.5,43.75 v45.25,43 58,43 59,44 J3.9
  Bottom 0.406: J3.9 64.99,44.01 65.12,43.88 74.71,43.88 X2.9 86.64,43.76 86.88,44 90.73,44 J1.9 100.33,43.98 X1.9
18  (via drill 0.7)
  Top 0.305: v45.25,45.25 42.5,42.5 40.65,42.5 R50.1
  Bottom 0.305: RN15.10 41.38,46.12 42.25,45.25 v45.25,45.25 61.09,45.25 J3.22
  Bottom 0.406: J3.22 62.09,45.41 62.38,45.12 77.64,45.12 X2.22 87.03,45.16 J1.28 99.62,45.38 99.88,45.12 X1.28
19  (via drill 0.7)
  Top 0.305: R51.1 42.75,43.75 44.25,45.25 v44.25,46.25
  Bottom 0.305: RN15.11 41.58,46.92 42.25,46.25 v44.25,46.25 59.62,46.25 60.12,46.75 64.72,46.75 J3.10
  Bottom 0.406: J3.10 74.58,46.78 X2.10 86.53,46.53 86.62,46.62 90.63,46.62 J1.10 100.33,46.75 X1.10
20  (via drill 0.7)
  Top 0.305: R52.1 42.12,45.12 43,46 v43,47.25
  Bottom 0.305: RN15.12 42.52,47.73 v43,47.25 59.62,47.25 60.5,48.12 61.22,48.12 J3.23
  Bottom 0.406: J3.23 61.4,48 75.25,48 75.35,47.9 X2.23 87.03,47.9 J1.29 99.38,48.12 99.62,47.88 X1.29
21  (via drill 0.7)
  Top 0.305: R53.1 40.75,46.5 42.5,48.25 v44,48.25
  Bottom 0.305: RN15.13 42.23,48.52 42.5,48.25 v44,48.25 59.25,48.25 60.5,49.5 64.7,49.5 J3.11
  Bottom 0.406: J3.11 74.58,49.55 X2.11 90.53,49.3 J1.11 100.33,49.52 X1.11
22  (via drill 0.7)
  Top 0.305: R54.1 41.5,48 v42.83,49.33
  Bottom 0.305: RN15.14 v42.83,49.33 59.2,49.33 60.75,50.88 61.2,50.88 J3.24
  Bottom 0.406: J3.24 73.95,50.92 74.12,50.75 77.59,50.75 X2.24 87.03,50.67 J1.30 99.61,50.89 99.75,50.75 103.31,50.75 X1.30
23  (via drill 0.7)
  Top 0.305: R55.1 41.5,49.5 v43.25,51.25
  Bottom 0.305: RN15.15 42.12,50.12 v43.25,51.25 59.25,51.25 60.25,52.25 64.71,52.25 J3.12
  Bottom 0.406: J3.12 65.71,52.29 65.88,52.12 74.75,52.12 X2.12 86.54,52.04 86.75,52.25 J1.12 100.33,52.26 X1.12
24  (via drill 0.7)
  Top 0.305: R56.1 41.5,51 v41.88,51.38
  Bottom 0.305: RN15.16 41.42,50.92 v41.88,51.38 43.25,52.75 59.12,52.75 60.12,53.75 61.19,53.75 J3.25
  Bottom 0.406: J3.25 61.31,53.75 65.75,53.75 66.06,53.44 X2.25 87.03,53.44 J1.31 98.97,53.66 99.25,53.38 103.39,53.38 X1.31
25  (via drill 0.7)
  Top 0.305: R57.1 41.75,52.75 v44.5,55.5
  Bottom 0.305: RN16.9 42.3,55.7 42.5,55.5 v44.5,55.5 64.31,55.5 J3.13
  Bottom 0.406: J3.13 74.58,55.06 X2.13 75.14,55.12 89.62,55.12 89.72,55.03 J1.13 100.33,55.03 X1.13
26  (via drill 0.7)
  Top 0.305: R58.1 41.75,54.25 v44.62,57.12
  Bottom 0.305: RN16.10 42.25,56.5 42.5,56.25 43.75,56.25 v44.62,57.12 86.52,57.12 J1.32
  Bottom 0.406: J1.32 99.6,56.4 99.88,56.12 103.39,56.12 X1.32
27  (via drill 0.7)
  Top 0.305: R59.1 41.7,55.75 v43.25,57.3
  Bottom 0.305: RN16.11 v43.25,57.3 43.42,57.3 44.38,58.25 85.25,58.25 85.75,57.75 90.7,57.75 J1.14
  Bottom 0.406: J1.14 100.33,57.8 X1.14
28  (via drill 0.7)
  Top 0.305: R60.1 41.5,57.25 v43.38,59.12
  Bottom 0.305: RN16.12 41.4,58.1 41.5,58 42.25,58 v43.38,59.12 74.5,59.12 74.88,58.75 86.83,58.75 J1.33
  Bottom 0.406: J1.33 99.7,59.17 99.88,59 103.34,59 X1.33
29  (via drill 0.7)
  Top 0.305: R61.1 41.75,58.75 v41.9,58.9
  Bottom 0.305: RN16.13 v41.9,58.9 43.12,60.12 57.62,60.12 62.25,64.75 78,64.75 82.38,60.38 90.58,60.38 J1.15
  Bottom 0.406: J1.15 99.46,60.54 99.62,60.38 100.5,60.38 X1.15
30  (via drill 0.7)
  Top 0.305: R62.1 42,60.25 v42.75,61
  Bottom 0.305: RN16.14 40.38,59.75 41.5,59.75 v42.75,61 57.62,61 61.88,65.25 78.62,65.25 82,61.88 87.18,61.88 J1.34
  Bottom 0.406: J1.34 99.44,61.94 99.75,61.62 103.36,61.62 X1.34
31  (via drill 0.7)
  Top 0.305: R63.1 40.52,61.77 v41.75,63
  Bottom 0.305: RN16.15 41,60.5 41.75,61.25 v41.75,63 58.75,63 61.5,65.75 79.12,65.75 81.62,63.25 90.69,63.25 J1.16
  Bottom 0.406: J1.16 100.33,63.31 X1.16
32  (via drill 0.7)
  Top 0.305: R64.1 40.52,64.8 v40.33,65
  Bottom 0.305: RN16.16 v40.33,65 60.12,65 61.38,66.25 79.62,66.25 81.25,64.62 87.19,64.62 J1.35
  Bottom 0.406: J1.35 99.44,64.68 99.62,64.5 103.36,64.5 X1.35
33  (via drill 0.7)
  Top 0.305: R65.1 v44.5,73
  Bottom 0.305: RN17.9 43.8,76.95 44.5,76.25 v44.5,73 45.12,72.38 45.12,69.5 47.88,66.75 80.25,66.75 81.12,65.88 90.55,65.88 J1.17
  Bottom 0.406: X1.17 91,65.83 J1.17
34  (via drill 0.7)
  Top 0.305: R66.1 v45.38,74.5
  Bottom 0.305: v45.38,74.5 45.38,76.12 43.75,77.75 RN17.10 | v45.38,74.5 45.38,74.25 | J1.36 87.05,67.25 86.5,67.25 80.5,73.25 46.62,73.25 v45.38,74.5
  Bottom 0.406: J1.36 99.55,67.45 99.75,67.25 103.37,67.25 X1.36
35  (via drill 0.7)
  Top 0.305: R67.1 v46.38,76
  Bottom 0.305: RN17.11 43.12,78.5 44,78.5 46.38,76.12 v46.38,76 48.62,73.75 81,73.75 85.88,68.88 90.7,68.88 J1.18
  Bottom 0.406: J1.18 100.33,68.82 X1.18
36  (via drill 0.7)
  Top 0.305: R68.1 v46.62,77.5
  Bottom 0.305: RN17.12 43.17,79.25 44.12,79.25 45.88,77.5 v46.62,77.5 46.75,77.5 46.75,76.88 49.38,74.25 84,74.25 87.15,71.1 87.15,70.12 J1.37
  Bottom 0.406: J1.37 99.66,70.22 99.88,70 103.39,70 X1.37
37  (via drill 0.7)
  Top 0.305: v46.88,79.25 R69.1
  Bottom 0.305: RN17.13 45.98,80.15 v46.88,79.25 46.88,78.75 50.88,74.75 86.5,74.75 89.66,71.59 J1.19
  Bottom 0.406: J1.19 100.33,71.59 X1.19
+5V  (via drill 0.7)
  Top 0.305: C5.2 25.02,22.23 25.25,22
  Top 0.406: R70.2 22.17,14.95 22.07,15.04
  Top 0.5: v26.5,22 25.25,22 23.5,22 v21.25,19.88
  Top 0.61: v25.75,78.75 25.75,79.75 27.5,81.5 30.24,81.5 C2.2 30.37,81.5 v34.5,81.5 39.6,81.5 R69.2 R68.2 R67.2 R66.2 R65.2 39.23,70.38 R64.2 R63.2 R62.2 R61.2 R60.2 R59.2 R58.2 R57.2 R56.2 R55.2 | v21.25,47 23.73,49.48 C6.2 25.02,49.5 v30.12,49.5 R55.2 | R55.2 R54.2 R53.2 R52.2 R51.2 R50.2 R49.2 39.25,40.98 39.25,40 37.85,38.6 R48.2 R47.2 R46.2 R45.2 R44.2 R43.2 R42.2 R41.2 R40.2 | R33.2 R34.2 R35.2 R36.2 R37.2 R38.2 R39.2 R40.2 | v36.5,25.88 37.73,25.88 R40.2 | U6.15 v181.25,54.74 v181.25,54.75 | U6.18 177.44,54.7 v177.5,54.75 | U6.9 174.91,45.53 v175.62,46.25 | U5.18 177.44,30.93 v176.5,31.88 | v174.88,63.62 174.91,63.66 U7.9 174.91,69.03 177.38,71.5 177.38,75.16 U7.18 177.44,76.32 178.12,77 179.38,77 | v175,17.62 175,20.43 U5.9 | 179.38,77 179.5,77 179.5,77.25 v180,77.75 | 180,75.25 U7.16 179.99,76.39 179.38,77
  Top 0.813: J9.3 J9.1 22.07,15.04 52.95,15.04 58,10 167.38,10 v175,17.62
  Bottom 0.406: U1.18 U1.17 23.61,77.5 22.5,77.5 22,77 22,75.5 22.5,75 U1.15 | U2.18 17.93,19.43 17.62,19.12 17.62,16.88 | 17.62,16.88 17.62,16.12 18.25,15.5 18.9,15.5 U2.15 | U2.16 17.64,16.89 17.62,16.88 | R71.2 4.67,14.95 6.47,13.15 9.38,13.15 J9.1
  Bottom 0.5: 32,25.88 29.62,23.5 29.62,22.75 28.84,21.97 U2.9 26.28,21.97 v26.5,22 | U2.18 20.93,19.43 v21.25,19.88
  Bottom 0.61: U1.9 34.34,81.34 v34.5,81.5 | U1.18 25.7,78.81 v25.75,78.75 | U3.9 30.09,49.47 v30.12,49.5 | v21.25,47 19.09,47 U3.18 U3.17 | 32,25.88 v36.5,25.88 | C7.2 181.25,50.73 v181.25,54.75 181.25,55.5 180.25,56.5 177.75,56.5 177.5,56.25 | v177.5,54.75 177.5,55.5 | v177.5,54.75 175.62,52.88 v175.62,46.25 175.62,41.5 177.44,39.68 177.44,31.93 | 177.44,31.93 U5.18 177.4,29.68 C8.2 177.4,25.02 175,22.62 v175,17.62 | 177.44,31.93 177.38,32 176.62,32 v176.5,31.88 | v174.88,63.62 174.88,63.5 177.5,60.88 177.5,56.25 | 177.5,56.25 v177.5,54.75 | C3.2 179.78,77.53 v180,77.75 | 17.62,16.88 13.1,16.88 J9.1
DSUB
  Bottom 0.305: RN13.1 35.45,19.07 35.25,18.88 35.25,12.38 33.88,11 24.12,11 22.12,13 22.12,21.75 20.64,23.24 U2.21
  Bottom 0.406: U2.21 19,23.23 16.9,23.23 12.53,18.85 10.05,18.85 8.79,17.59 J9.4 8.02,16.88 R71.1
GND  (via drill 0.7)
  Top 0.305: C5.1 24.35,20.52 24.25,20.62
  Top 0.61: v35,79.5 30.54,79.5 C2.1 30.2,79.62 28.5,79.62 v25.88,77 | v30.25,47.75 25.02,47.75 | 25.02,47.75 C6.1 | 25.02,47.75 24.5,47.75 v21.25,44.5 | v179.75,54.75 179.99,54.52 U6.16 U6.17 | U6.10 176.18,44.55 v177.62,46 | U5.17 178.72,31.84 v178.75,31.88 180.75,31.88 181.25,31.37 U5.15 U5.16 | v177.5,63.62 176.18,64.95 U7.10 176.18,68.55 178.88,71.25 178.88,73.62 | v176.88,17.5 176.88,18.12 176.12,18.88 176.12,20.47 U5.10 | 178.88,73.62 178.88,75.07 U7.17 | 178.88,73.62 179,73.5 181,73.5 181.25,73.75 U7.15 181.25,77.62 v181.38,77.75 | v26.5,20.62 24.25,20.62 23.88,20.62 v21.25,18 21.23,18.02
  Top 0.813: J9.7 12.84,22.66 17.38,18.12 21.12,18.12 v21.25,18 | J9.7 J9.9 | J9.7 J9.8 J9.10
  Bottom 0.406: U2.10 30.57,20.7 v30.62,20.75
  Bottom 0.61: U1.10 34.42,80.08 v35,79.5 | U3.10 29.8,48.2 v30.25,47.75 | v21.25,44.5 19.13,44.5 U3.16 U3.15 | U2.10 26.57,20.7 v26.5,20.62 | v179.75,54.75 179.75,50.52 C7.1 177.62,48.1 v177.62,46 | v177.62,46 177.62,41.25 178.75,40.12 v178.75,31.88 178.75,27.1 C8.1 179.1,24.85 176.88,22.62 v176.88,17.5 | v177.5,63.62 177.5,62.38 179.25,60.62 179.25,58.38 179.88,57.75 180.5,57.75 183,55.25 183,49 180,46 v177.62,46 | C3.1 181.47,77.65 v181.38,77.75 | U1.16 25.14,76.27 v25.88,77 | U2.17 21.09,18.16 v21.25,18
  Bottom 1.27: J9.9 11.27,38.52 15.75,43 18.9,43 U3.15
  pour Top (isolate 0.813): 0.75,123 195.5,123 195.5,1.5 0.75,1.5
N$2
  Bottom 0.305: U2.22 20.36,24.51 22.62,22.25 22.62,13.38 24.5,11.5 33.5,11.5 34.62,12.62 34.62,19.62 34.88,19.88 RN13.2
N$3
  Bottom 0.305: U2.23 20.72,25.78 21,25.5 21,24.62 23.12,22.5 23.12,13.75 24.88,12 32.88,12 34.12,13.25 34.12,20.5 34.38,20.75 37.65,20.75 RN13.3
N$4
  Bottom 0.305: U2.24 21.07,27.05 21.5,26.62 21.5,24.88 23.62,22.75 23.62,13.88 25,12.5 32.38,12.5 33.62,13.75 33.62,21.12 34,21.5 37.7,21.5 RN13.4
N$5
  Bottom 0.305: U2.25 21.8,28.32 22,28.12 22,25.12 24.12,23 24.12,14.12 25.25,13 32,13 33,14 33,21.88 33.38,22.25 37.7,22.25 RN13.5
N$6
  Bottom 0.305: U2.26 22.16,29.59 22.5,29.25 22.5,25.38 24.62,23.25 24.62,14.5 25.5,13.62 31.75,13.62 32.5,14.38 32.5,22.62 33,23.12 37.67,23.12 RN13.6
N$7
  Bottom 0.305: U2.27 22.64,30.86 23,30.5 23,25.88 25.12,23.75 25.12,14.88 25.88,14.12 31.25,14.12 32,14.88 32,23 33,24 37.6,24 RN13.7
N$8
  Bottom 0.305: U2.28 23.12,32.13 23.5,31.75 23.5,26.12 25.62,24 25.62,15.25 26.25,14.62 30.88,14.62 31.5,15.25 31.5,23.38 32.75,24.62 37.67,24.62 RN13.8
N$9
  Bottom 0.305: U3.21 19.89,50.74 22.5,48.12 22.5,40.62 24.75,38.38 32.62,38.38 35.62,41.38 35.75,41.38 39,44.62 39,45.23 RN15.1 39.02,45.25
N$10
  Bottom 0.305: U3.22 20.24,52.01 20.5,51.75 20.5,51 23.12,48.38 23.12,40.88 25.12,38.88 32.25,38.88 38.25,44.88 38.25,45.62 38.75,46.12 RN15.2
N$11
  Bottom 0.305: U3.23 20.72,53.28 21,53 21,51.38 23.62,48.75 23.62,41.25 25.5,39.38 31.75,39.38 37.62,45.25 37.62,46.12 38.5,47 39.02,47 RN15.3
N$12
  Bottom 0.305: U3.24 21.32,54.55 21.5,54.38 21.5,51.62 24.12,49 24.12,41.5 25.75,39.88 31.5,39.88 37,45.38 37,46.25 38.5,47.75 39.08,47.75 RN15.4
N$13
  Bottom 0.305: U3.25 21.68,55.82 22,55.5 22,51.88 24.75,49.12 24.75,41.75 26.12,40.38 31.12,40.38 36.38,45.62 36.38,46.62 38.25,48.5 39.08,48.5 RN15.5
N$14
  Bottom 0.305: U3.26 22.04,57.09 22.5,56.62 22.5,52.5 25.38,49.62 25.38,42 26.38,41 30.88,41 32.62,42.75 32.75,42.75 35.88,45.88 35.88,46.88 38.38,49.38 39.05,49.38 RN15.6
N$15
  Bottom 0.305: U3.27 22.77,58.36 23,58.12 23,52.75 25.88,49.88 25.88,42.25 26.62,41.5 30.62,41.5 35.25,46.12 35.25,47 38.38,50.12 RN15.7
N$16
  Bottom 0.305: U3.28 22.87,59.63 23.5,59 23.5,53.12 26.38,50.25 26.38,42.62 27,42 30.25,42 34.62,46.38 34.62,47.12 38.5,51 39.02,51 RN15.8
N$28
  Bottom 0.305: U1.21 25.64,82.61 27.75,80.5 27.75,71.75 30,69.5 37.5,69.5 40.5,72.5 40.5,76.75 40.75,77 41.67,77 RN17.1
N$30
  Bottom 0.305: U1.22 25.11,83.89 28.25,80.75 28.25,72.25 30.5,70 37.25,70 40,72.75 40,77.25 40.5,77.75 RN17.2
N$31
  Bottom 0.305: U1.23 25.09,85.16 25.5,84.75 25.5,84.25 29,80.75 29,72.5 30.75,70.75 37.25,70.75 39.5,73 39.5,78.25 39.75,78.5 41.67,78.5 RN17.3
N$32
  Bottom 0.305: U1.24 25.07,86.42 26,85.5 26,84.5 29.5,81 29.5,72.75 31,71.25 37,71.25 39,73.25 39,79 39.25,79.25 41.62,79.25 RN17.4
N$33
  Bottom 0.305: U1.25 25.8,87.69 26.5,87 26.5,84.75 30,81.25 30,73 31.25,71.75 36.75,71.75 38.5,73.5 38.5,79.75 39,80.25 41.62,80.25 RN17.5
PA0_5
  Top 0.305: U5.21 173.63,29.14 169.75,25.25 160.25,25.25 158.5,23.5 155.17,23.5 X5.1
  Top 0.406: J6.1 113.85,96.1 108.25,90.5 108.25,31 113.5,25.75 115.19,25.75 J4.1
  Bottom 0.406: J4.1 X6.1 128.39,23 132.12,23 132.41,23.28 J2.1 154.95,23.28 X5.1 | J6.1 X7.1 130.98,96.1 140,105.12 141.97,105.12 X8.1 J8.1
PA0_6
  Top 0.305: U6.21 173.63,51.88 170,48.25 161.75,48.25 159,45.5 155.1,45.5 X5.9
  Bottom 0.406: J4.9 X6.9 131.75,45 132.11,45.36 J2.9 146.38,45.48 X5.9
PA0_7
  Top 0.305: U7.21 173.63,74.39 170.62,71.38 162.75,71.38 159,67.62 155.12,67.62 X5.17
  Bottom 0.406: J2.17 154.95,67.45 X5.17
PA1_5
  Top 0.305: U5.22 172.37,28.99 169.12,25.75 158.89,25.75 X5.20
  Top 0.406: J4.14 113.69,24.31 107.5,30.5 107.5,91.75 113.25,97.5 115,97.5 J6.9
  Bottom 0.406: J4.14 X6.14 131.24,24.38 132.5,24.38 132.78,24.66 J2.20 153.91,24.66 154,24.75 157.89,24.75 X5.20 | J6.9 X7.9 131.35,94.73 140.5,103.88 144.91,103.88 X8.6 J8.6
PA1_6
  Top 0.305: U6.22 172.37,51.62 169.5,48.75 160.5,48.75 158.75,47 158.04,47 X5.28
  Bottom 0.406: J4.22 X6.22 131.52,46.75 J2.28 142.75,46.75 147.12,46.75 147.25,46.88 X5.28
PA1_7
  Top 0.305: U7.22 172.37,74.49 169.75,71.88 161.25,71.88 158.5,69.12 158.1,69.12 X5.36
  Bottom 0.406: J2.36 154.2,68.83 154.38,69 157.87,69 X5.36
PA2_5
  Top 0.305: U5.23 171.09,29.34 168,26.25 155.18,26.25 X5.2
  Top 0.406: J6.2 113.86,93.36 109.75,89.25 109.75,32 113.25,28.5 115.21,28.5 J4.2
  Bottom 0.406: J4.2 X6.2 128.37,25.75 132.25,25.75 132.53,26.03 J2.2 146.38,26.15 X5.2 | J6.2 X7.2 131.36,93.36 140.62,102.62 141.95,102.62 X8.2 J8.2
PA2_6
  Top 0.305: U6.23 171.09,51.84 168.5,49.25 159.75,49.25 158.75,48.25 X5.10
  Bottom 0.406: J4.10 X6.10 128.36,47.75 132.38,47.75 132.75,48.12 J2.10 146.38,48.25 X5.10
PA2_7
  Top 0.305: U7.23 171.09,74.59 168.88,72.38 160.62,72.38 158.62,70.38 155.13,70.38 X5.18
  Bottom 0.406: J2.18 154.95,70.2 X5.18
PA3_5
  Top 0.305: U5.24 169.82,29.2 167.38,26.75 162.25,26.75 161.25,27.75 158.12,27.75 X5.21
  Top 0.406: J4.15 113.67,27.08 109,31.75 109,90.25 113.5,94.75 115.01,94.75 J6.10
  Bottom 0.406: J4.15 X6.15 131.22,27.12 132.25,27.12 132.55,27.42 J2.21 142.87,27.55 X5.21 | J6.10 X7.10 131.74,91.99 140.88,101.12 X8.7 J8.7
PA3_6
  Top 0.305: U6.24 169.82,51.83 167.75,49.75 158.05,49.75 X5.29
  Bottom 0.406: J4.23 X6.23 131.52,49.5 J2.29 142.87,49.62 X5.29
PA3_7
  Top 0.305: U7.24 169.82,74.58 168.12,72.88 159.08,72.88 X5.37
  Bottom 0.406: J2.37 143.72,71.59 143.88,71.75 157.89,71.75 X5.37
PA4_5
  Top 0.305: U5.25 168.56,29.3 166.5,27.25 162.62,27.25 160.88,29 155.16,29 X5.3
  Top 0.406: J6.3 113.36,90.61 111.25,88.5 111.25,32.75 112.75,31.25 115.2,31.25 J4.3
  Bottom 0.406: J4.3 X6.3 128.4,28.38 132.25,28.38 132.67,28.8 J2.3 146.38,28.92 X5.3 | J6.3 X7.3 131.87,90.61 141,99.75 X8.3 J8.3
PA4_6
  Top 0.305: U6.25 168.56,52.05 166.75,50.25 161.75,50.25 161,51 155.1,51 X5.11
  Bottom 0.406: J4.11 X6.11 128.38,50.5 131.88,50.5 132.27,50.89 J2.11 146.38,51.02 X5.11
PA4_7
  Top 0.305: U7.25 168.56,74.18 167.75,73.38 155.36,73.38 X5.19
  Bottom 0.406: J2.19 154.95,72.97 X5.19
PA5_5
  Top 0.406: J4.16 112.9,29.85 110.5,32.25 110.5,89 113.5,92 114.75,92 116.25,90.5 116.52,90.5 J6.11 | U5.26 167.28,29.04 166,27.75 163.12,27.75 160.5,30.38 158,30.38 X5.22
  Bottom 0.406: J4.16 X6.16 131.2,29.88 132.25,29.88 132.54,30.17 J2.22 142.87,30.29 X5.22 | J6.11 X7.11 132.12,89.24 141.25,98.38 X8.8 J8.8
PA5_6
  Top 0.305: U6.26 167.28,52.03 166,50.75 162,50.75 160.25,52.5 158.03,52.5 X5.30
  Bottom 0.406: J4.24 130.62,51.92 | 130.62,51.92 X6.24 | 130.62,51.92 130.97,52.27 J2.30 142.87,52.39 X5.30
PA6_5
  Top 0.305: 166.01,28.77 165.62,28.38 163.75,28.38
  Top 0.406: J6.4 114.12,87.87 112.75,86.5 112.75,34.25 113,34 115.75,34 117,32.75 117,32.22 J4.4 | U5.27 166.01,28.77 | 163.75,28.38 160.38,31.75 155.14,31.75 X5.4
  Bottom 0.406: J4.4 X6.4 128.42,31.12 132.38,31.12 132.81,31.56 J2.4 146.38,31.69 X5.4 | J6.4 X7.4 132.12,87.87 141,96.75 141.82,96.75 X8.4 J8.4
PA6_6
  Top 0.305: U6.27 166.01,51.52 165.75,51.25 162.5,51.25 160,53.75 X5.12
  Bottom 0.406: J4.12 X6.12 128.37,53.25 131.88,53.25 132.26,53.64 J2.12 154.95,53.64 X5.12
PA7_5
  Top 0.406: J6.12 117.75,86.5 115,89.25 113.5,89.25 112,87.75 112,33.5 113,32.5 114.41,32.5 J4.17 | U5.28 163.77,29.73 160.25,33.25 158.11,33.25 X5.23
  Bottom 0.406: J4.17 X6.17 131.52,32.94 J2.23 142.87,33.06 X5.23 | J6.12 X7.12 132.25,86.5 141.38,95.62 144.91,95.62 X8.9 J8.9
PA7_6
  Top 0.305: U6.28 162.4,52.6 159.75,55.25 158.01,55.25 X5.31
  Bottom 0.406: J4.25 X6.25 131.52,55.03 J2.31 157.8,55.03 X5.31
PB0_1
  Bottom 0.305: U2.1 29.37,32.13 32.5,29 37.8,29 RN14.1
PB0_2
  Bottom 0.305: U3.1 30.37,59.63 34.38,55.62 38.9,55.62 RN16.1
PB0_5
  Top 0.305: U5.1 164.75,21.87 167.62,24.75 170.62,24.75 174.12,28.25 184.38,28.25 185.62,29.5 185.62,31.75 182.88,34.5 155.15,34.5 X5.5
  Bottom 0.406: X5.5 154.95,34.31 J2.5 132.18,34.31 131.88,34 X6.5 J4.5 112.5,34 107.5,39 107.5,79.25 113.38,85.13 J6.5 X7.5 132.94,85.13 X8.5 J8.5
PB0_6
  Top 0.305: X5.13 155.11,56.5 158.5,56.5 159,56 183.5,56 185.75,53.75 185.75,52 184.75,51 173.75,51 170.5,47.75 168.5,47.75 165.25,44.5 165,44.5 164.75,44.25 U6.1
  Bottom 0.406: J4.13 X6.13 128.67,56.41 J2.13 154.95,56.41 X5.13
PB1_1
  Bottom 0.305: U2.2 27.39,30.86 27,31.25 27,32.75 27.12,32.88 29.75,32.88 32.88,29.75 RN14.2
PB1_2
  Bottom 0.305: U3.2 27.27,58.36 27,58.62 27,60.25 27.12,60.38 30.38,60.38 34.38,56.38 38.85,56.38 RN16.2
PB1_5
  Top 0.305: U5.2 166.01,22.27 168,24.25 171.25,24.25 174.62,27.62 184.62,27.62 186.38,29.38 186.38,31.75 183.12,35 158.75,35 X5.24
  Bottom 0.406: X5.24 157.8,35.7 J2.24 132.7,35.7 132.38,35.38 131.19,35.38 X6.18 J4.18 114.36,35.5 112.25,35.5 108.25,39.5 108.25,79 113.01,83.76 J6.13 X7.13
PB1_6
  Top 0.305: X5.32 159.07,56.75 184,56.75 186.5,54.25 186.5,51.75 185.25,50.5 174,50.5 170.75,47.25 169.25,47.25 166,44 166,43.41 U6.2
  Bottom 0.406: J2.32 157.8,57.78 X5.32
PB2_1
  Bottom 0.305: U2.3 27.41,29.59 26.5,30.5 26.5,32.88 27,33.38 30,33.38 32.88,30.5 37.8,30.5 RN14.3
PB2_2
  Bottom 0.305: U3.3 27.29,57.09 26.5,57.88 26.5,60.38 27,60.88 30.62,60.88 34.25,57.25 38.92,57.25 RN16.3
PB2_5
  Top 0.305: U5.3 167.28,22.29 168.75,23.75 171.62,23.75 175,27.12 184.88,27.12 186.88,29.12 186.88,32 183.38,35.5 162.75,35.5 161.12,37.12 155.75,37.12 155.62,37.25 155.13,37.25 X5.6
  Bottom 0.406: X5.6 146.38,37.2 J2.6 132.58,37.08 132.12,36.62 128.43,36.62 X6.6 J4.6 117.98,36.75 112.75,36.75 109,40.5 109,78.75 112.64,82.39 J6.6 X7.6
PB2_6
  Top 0.305: X5.14 155.13,59.25 158.5,59.25 160.25,57.5 184.25,57.5 187.25,54.5 187.25,51.75 185.5,50 174.25,50 171,46.75 169.75,46.75 167.5,44.5 167.5,43.61 U6.3
  Bottom 0.406: J2.14 154.95,59.17 X5.14
PB3_1
  Bottom 0.305: U2.4 27.3,28.32 26,29.62 26,33.25 26.62,33.88 30.38,33.88 32.88,31.38 37.83,31.38 RN14.4
PB3_2
  Bottom 0.305: U3.4 27.3,55.82 26,57.12 26,60.75 27.12,61.88 30.5,61.88 34.25,58.12 38.95,58.12 RN16.4
PB3_5
  Top 0.305: U5.4 168.56,22.18 169.62,23.25 172.12,23.25 175.5,26.62 185.12,26.62 187.62,29.12 187.62,32 183.5,36.12 162.88,36.12 160.5,38.5 158.02,38.5 X5.25
  Bottom 0.406: X5.25 147.47,38.6 147.38,38.5 142.77,38.5 J2.25 133.1,38.47 132.75,38.12 X6.19 J4.19 114.38,38.25 113,38.25 109.75,41.5 109.75,78.25 112.51,81.01 J6.14 X7.14
PB3_6
  Top 0.305: X5.33 158.09,60.5 158.5,60.5 160.75,58.25 184.5,58.25 187.75,55 187.75,51.5 185.75,49.5 174.5,49.5 171.25,46.25 170.75,46.25 168.75,44.25 168.75,43.59 U6.4
  Bottom 0.406: J2.33 157.8,60.55 X5.33
PB4_1
  Bottom 0.305: U2.5 27.32,27.05 25.5,28.88 25.5,33.5 26.38,34.38 30.62,34.38 33,32 37.7,32 RN14.5
PB4_2
  Bottom 0.305: U3.5 27.57,54.55 25.5,56.62 25.5,61 26.88,62.38 30.88,62.38 34.38,58.88 38.95,58.88 RN16.5
PB4_3
  Bottom 0.305: U1.5 32.08,86.42
PB4_5
  Top 0.305: U5.5 169.82,22.32 170.25,22.75 172.5,22.75 175.88,26.12 185.38,26.12 188.12,28.88 188.12,32.25 183.75,36.62 163.38,36.62 160,40 155.11,40 X5.7
  Bottom 0.406: X5.7 146.38,39.97 J2.7 132.59,39.84 132.25,39.5 X6.7 J4.7 113.25,39.5 110.5,42.25 110.5,77.5 112.64,79.64 J6.7 X7.7
PB4_6
  Top 0.305: X5.15 155.12,62 158.75,62 161.75,59 184.75,59 188.5,55.25 188.5,51.25 186.25,49 174.75,49 169.82,44.08 U6.5
  Bottom 0.406: J2.15 154.95,61.92 X5.15
PB5_1
  Bottom 0.305: U2.6 27.22,25.78 25,28 25,33.88 26,34.88 31.12,34.88 33,33 37.8,33 RN14.6
PB5_2
  Bottom 0.305: U3.6 27.59,53.28 25,55.88 25,61.25 26.62,62.88 31.12,62.88 34.25,59.75 38.92,59.75 RN16.6
PB5_3
  Bottom 0.305: U1.6 32.34,85.16
PB5_5
  Top 0.305: U5.6 171.09,21.72 171.62,22.25 172.75,22.25 176.12,25.62 185.62,25.62 188.62,28.62 188.62,32.62 184.12,37.12 163.75,37.12 159.62,41.25 158.01,41.25 X5.26
  Bottom 0.406: X5.26 142.87,41.34 J2.26 133.09,41.22 132.88,41 131.3,41 X6.20 J4.20 114.38,40.75 113.25,40.75 111.5,42.5 111.5,77.25 112.52,78.27 J6.15 X7.15
PB5_6
  Top 0.305: U6.6 171.09,44.59 175,48.5 186.75,48.5 189,50.75 189,55.5 185,59.5 162.25,59.5 158.75,63 158.36,63 X5.34
  Bottom 0.406: J2.34 157.8,63.31 X5.34
PB6_1
  Bottom 0.305: U2.7 27.24,24.51 24.5,27.25 24.5,34 25.88,35.38 31.5,35.38 33.25,33.62 37.73,33.62 RN14.7
PB6_2
  Bottom 0.305: U3.7 27.11,52.01 24.5,54.62 24.5,61.5 26.38,63.38 31.5,63.38 34.38,60.5 RN16.7
PB6_5
  Top 0.305: U5.7 172.37,21.49 172.62,21.75 173,21.75 176.38,25.12 185.88,25.12 189.12,28.38 189.12,33 184.5,37.62 164.38,37.62 159.38,42.62 158.75,42.62 158.64,42.74 X5.8
  Bottom 0.406: X5.8 146.38,42.74 J2.8 133.11,42.61 132.75,42.25 128.35,42.25 X6.8 J4.8 117.98,42.25 113.5,42.25 112.5,43.25 112.5,75.5 113.9,76.9 J6.8 X7.8
PB6_6
  Top 0.305: U6.7 172.37,45.12 175.25,48 187.25,48 189.5,50.25 189.5,56 185.25,60.25 163,60.25 158.5,64.75 155.14,64.75 X5.16
  Bottom 0.406: J2.16 154.95,64.69 X5.16
PB7_1
  Bottom 0.305: U2.8 27.51,23.24 24,26.75 24,34.25 25.62,35.88 31.88,35.88 33.25,34.5 37.8,34.5 RN14.8
PB7_2
  Bottom 0.305: U3.8 26.89,50.74 24,53.62 24,61.88 26,63.88 32.12,63.88 34.75,61.25 38.92,61.25 RN16.8
PB7_5
  Top 0.305: U5.8 173.63,21.64 176.62,24.62 186.25,24.62 189.75,28.12 189.75,33.12 184.75,38.12 164.75,38.12 158.75,44.12 157.94,44.12 X5.27
  Bottom 0.406: J4.21 X6.21 131.52,43.98 J2.27 153.99,43.98 154.12,44.12 157.91,44.12 X5.27
PB7_6
  Top 0.305: U6.8 173.63,45.63 175.5,47.5 187.5,47.5 190,50 190,56.25 185.25,61 163.25,61 158.5,65.75 158.35,65.75 X5.35
  Bottom 0.406: J2.35 157.8,66.06 X5.35
SCL1  (via drill 0.7)
  Top 0.406: U5.12 178.72,22.21 v180.25,23.75 | v180.25,40.12 178.75,41.62 178.75,43.36 U6.12 178.72,45.72 179.75,46.75 188,46.75 190.88,49.62 190.88,56.62 185.75,61.75 180,61.75 178.88,62.88 178.88,63 178.75,63.12 178.75,65.98 U7.12 | v31.38,53.38 31.38,77.25 v31.12,77.5 | v26.5,18.5 23.75,18.5 22.25,17 16.5,17 12.12,21.38 9.98,21.38 J9.6 7.38,21.48 7.38,28.25 24.75,45.62 v30.12,45.62
  Top 0.61: U7.12 178.72,68.84 180,70.12 v184.5,70.12
  Bottom 0.406: v180.25,23.75 v180.25,40.12 | v31.38,53.38 31.38,46.5 30.54,45.66 U3.12 30.09,45.66 v30.12,45.62 | v31.12,77.5 32.82,77.5 U1.12 | U2.12 26.84,18.16 v26.5,18.5
  Bottom 0.61: U1.12 35.16,77.53 36.12,78.5 36.12,105.38 44.75,114 138.5,114 140.25,115.75 164.12,115.75 187.12,92.75 187.12,72.75 v184.5,70.12
SDA1  (via drill 0.7)
  Top 0.406: U5.13 179.99,21.98 v181.62,23.62 | v181.62,40.12 181.62,40.25 180,41.88 U6.13 179.99,45.36 180.75,46.12 188.5,46.12 191.75,49.38 191.75,56.88 186.12,62.5 180.38,62.5 180,62.88 180,66 U7.13 | v32.62,53.5 32.62,74.38 v34.62,76.38 | v26.5,16.88 25.88,16.25 24.62,16.25 | 24.62,16.25 15.14,16.25 J9.5 10.02,18.88 7.75,18.88 6.62,20 6.62,28.5 24.75,46.62 32.12,46.62 32.38,46.88 v32.62,46.88 | R70.1 24.3,16.57 24.62,16.25
  Top 0.61: v180.12,68.12 180.12,66.16 U7.13
  Bottom 0.406: v181.62,23.62 v181.62,40.12 | 30.89,44.39 U3.13 30.23,44.39 30.25,44.38 30.88,44.38 30.89,44.39 | v32.62,53.5 v32.62,46.88 32.62,46.12 30.89,44.39 | v34.62,76.38 32.97,76.38 U1.13 | U2.13 26.52,16.89 v26.5,16.88
  Bottom 0.61: v34.62,76.38 35.62,76.38 37.12,77.88 37.12,101.62 42,106.5 137.5,106.5 138.75,107.75 170,107.75 185.88,91.88 185.88,73.88 v180.12,68.12

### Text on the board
tPlace: FEMALE | FEMALE | FEMALE | FEMALE | RADIOSCH.EU | FEMALE | FEMALE | FEMALE | FEMALE
bPlace: RADIOSCH.EU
